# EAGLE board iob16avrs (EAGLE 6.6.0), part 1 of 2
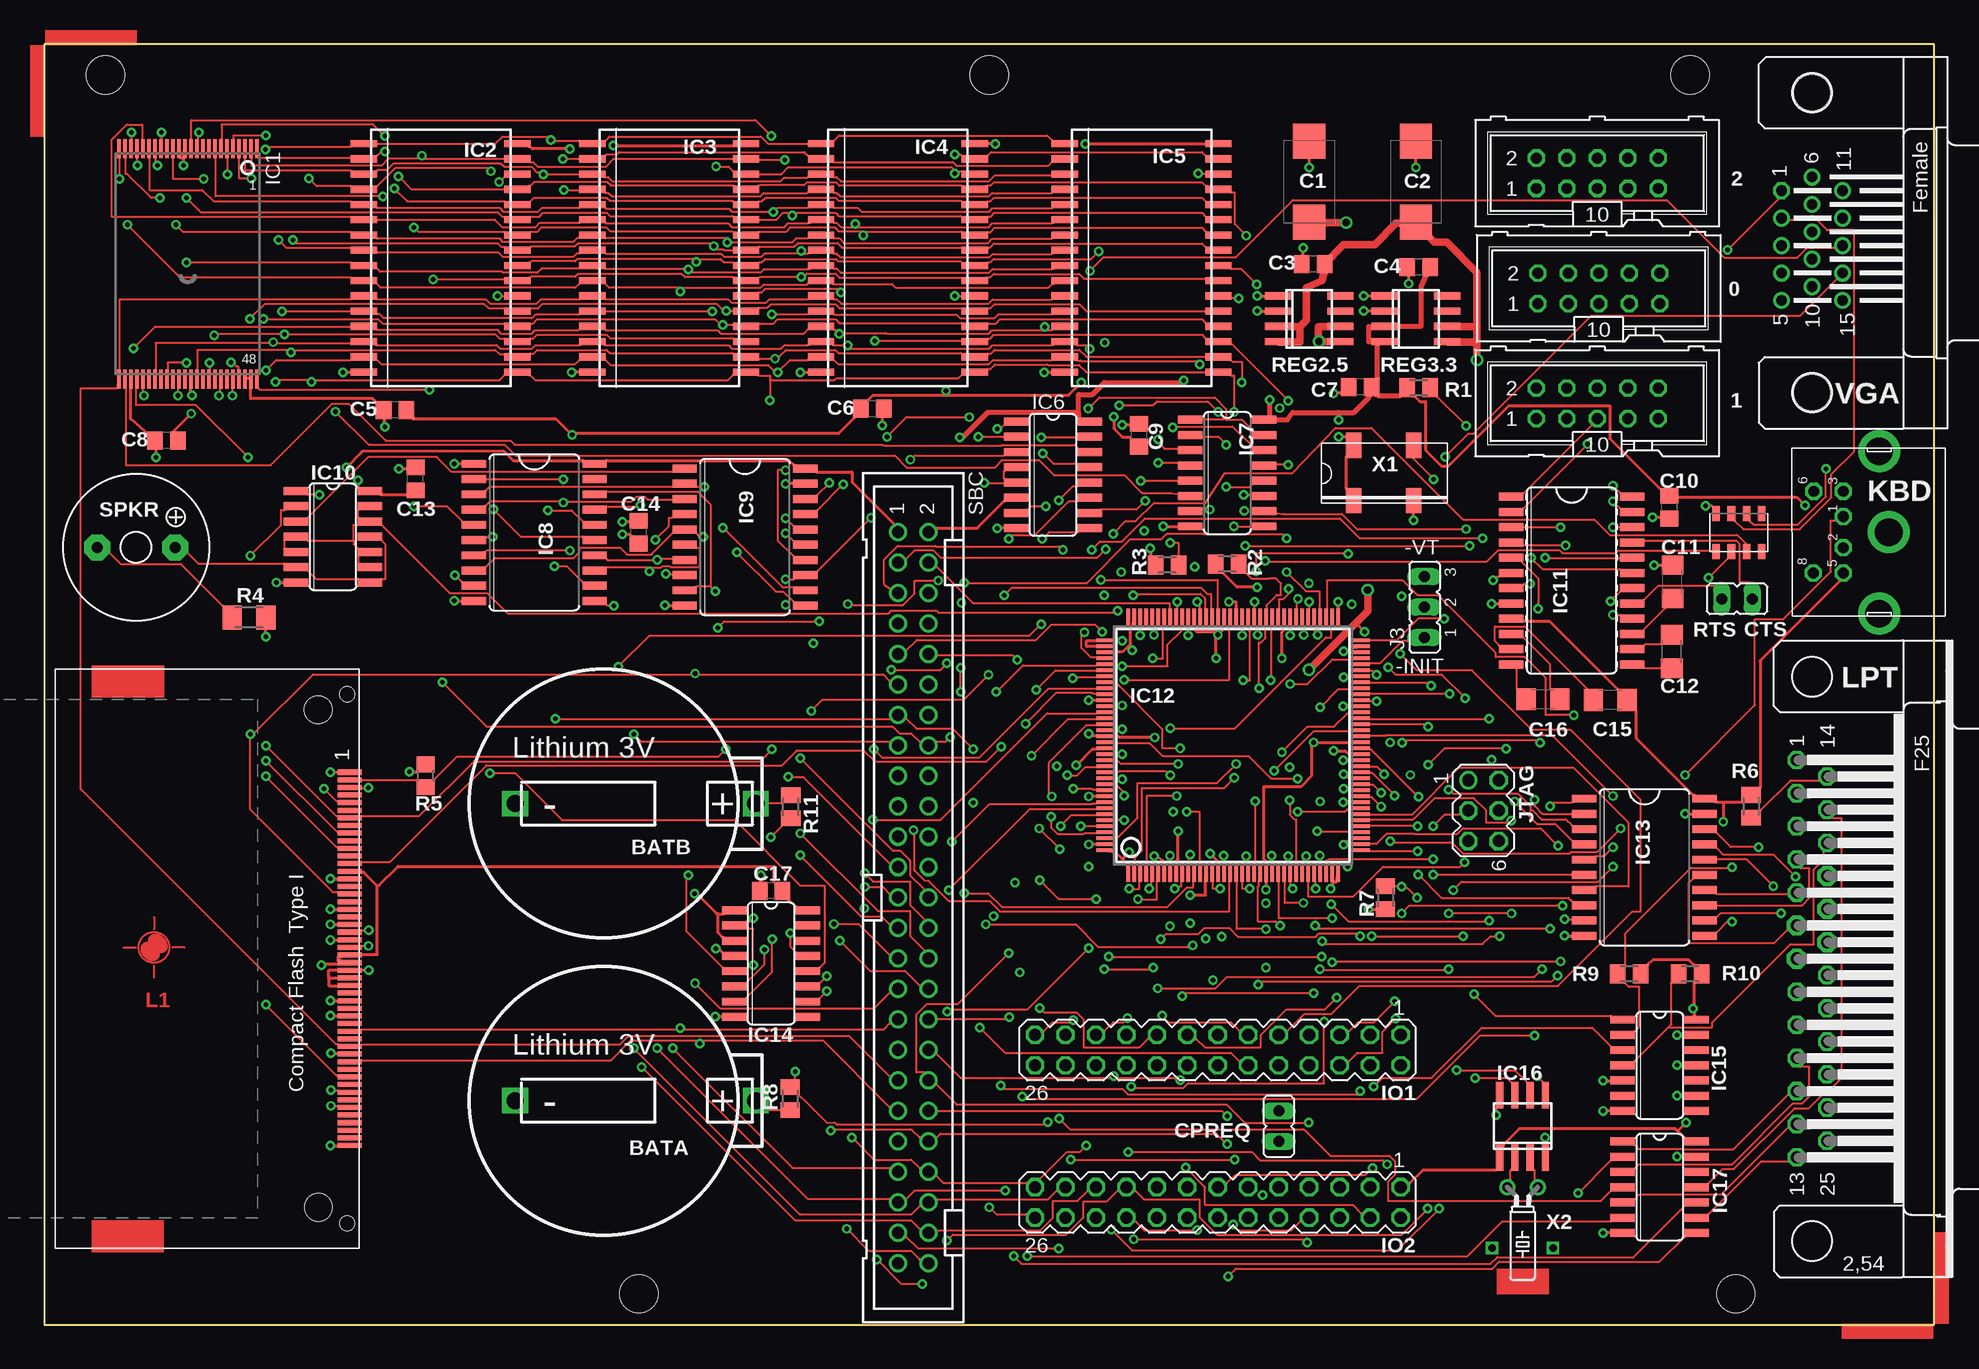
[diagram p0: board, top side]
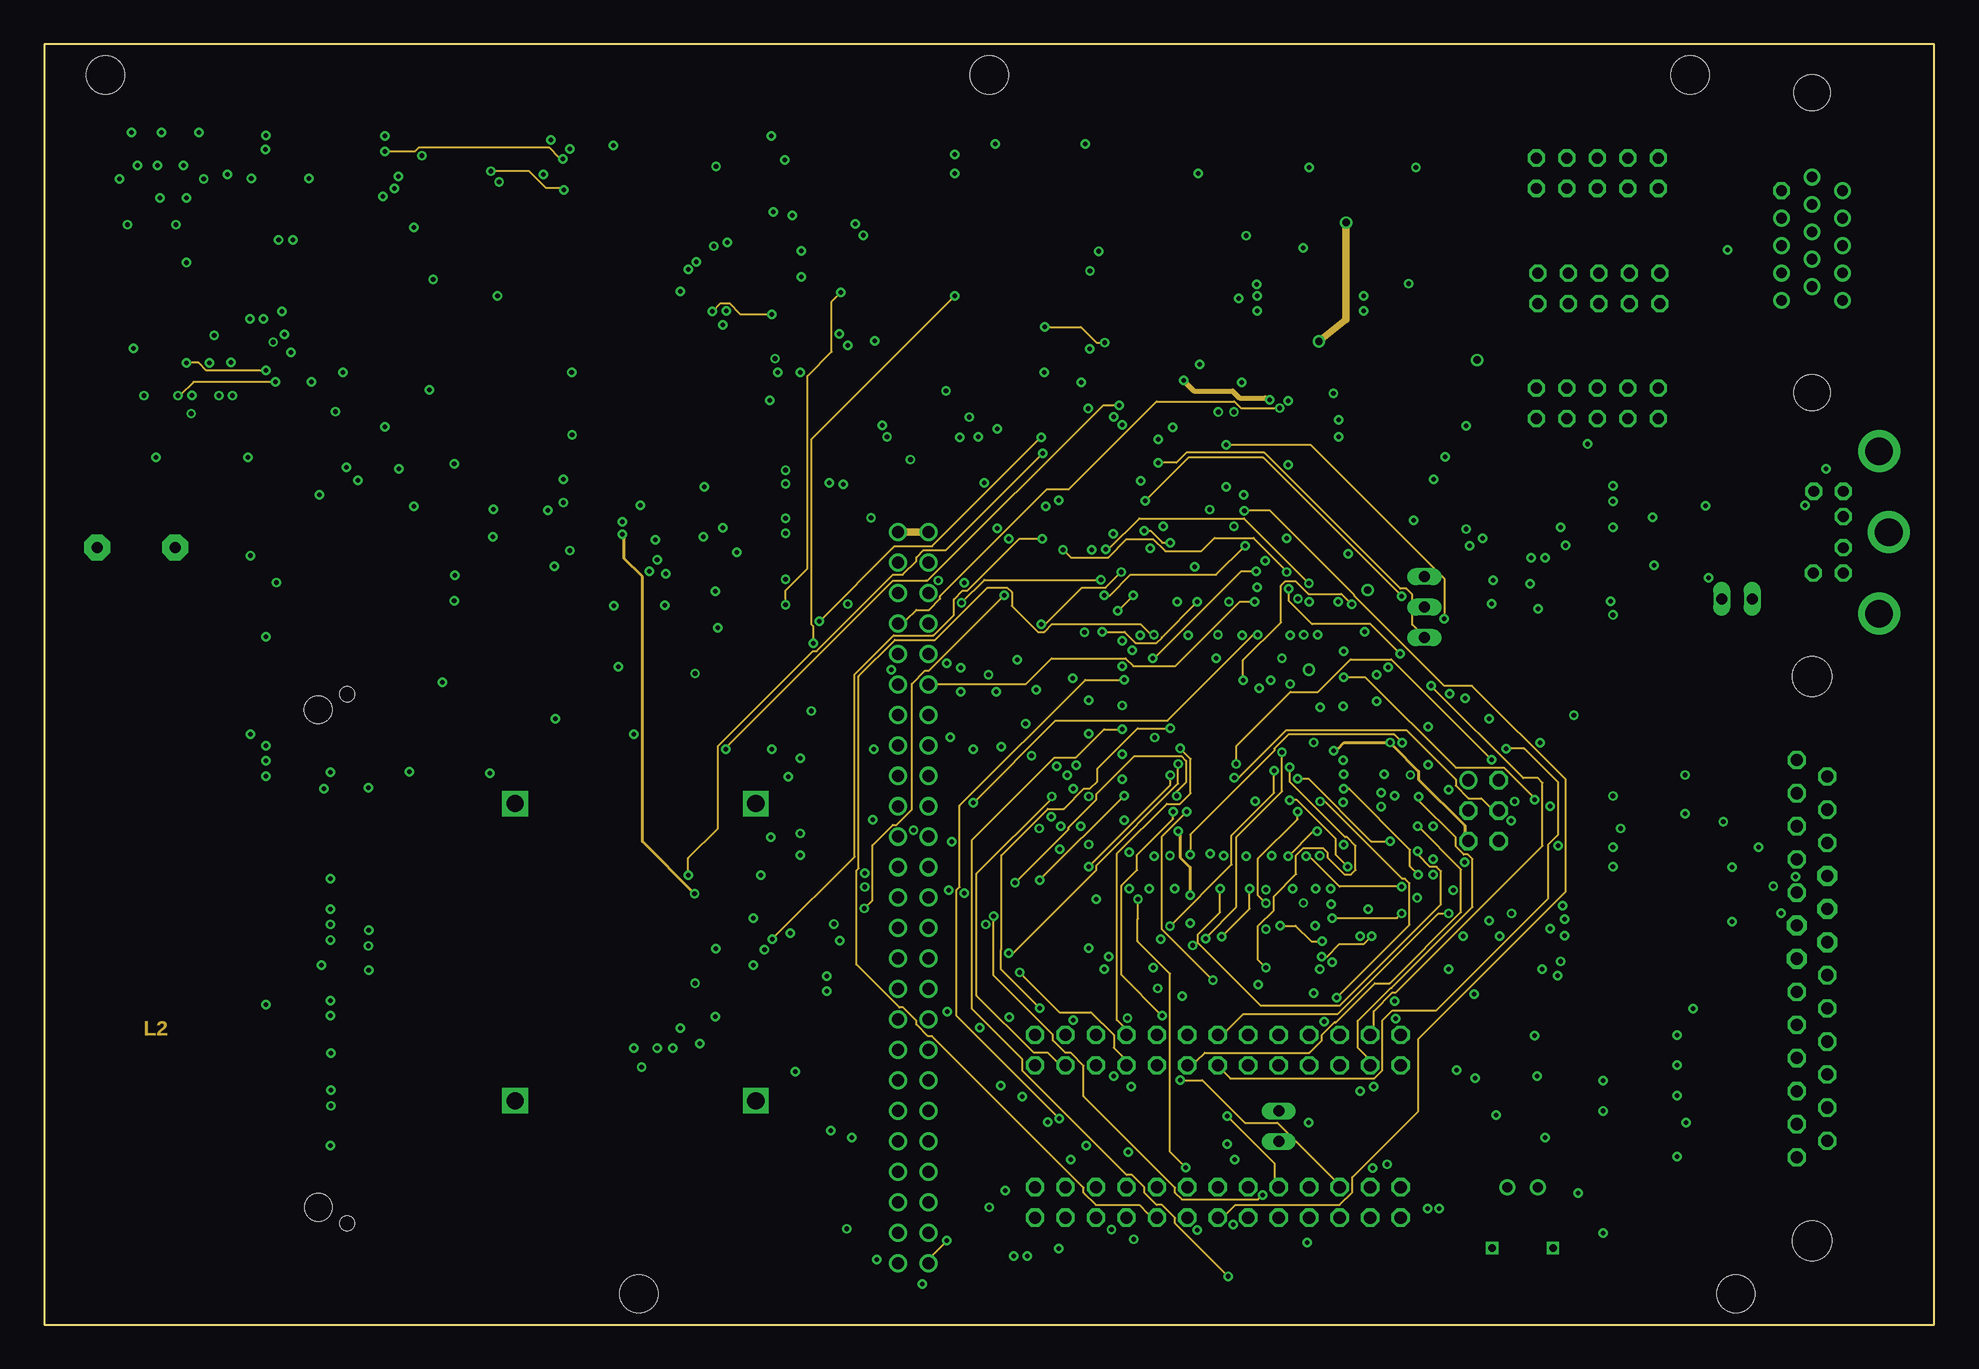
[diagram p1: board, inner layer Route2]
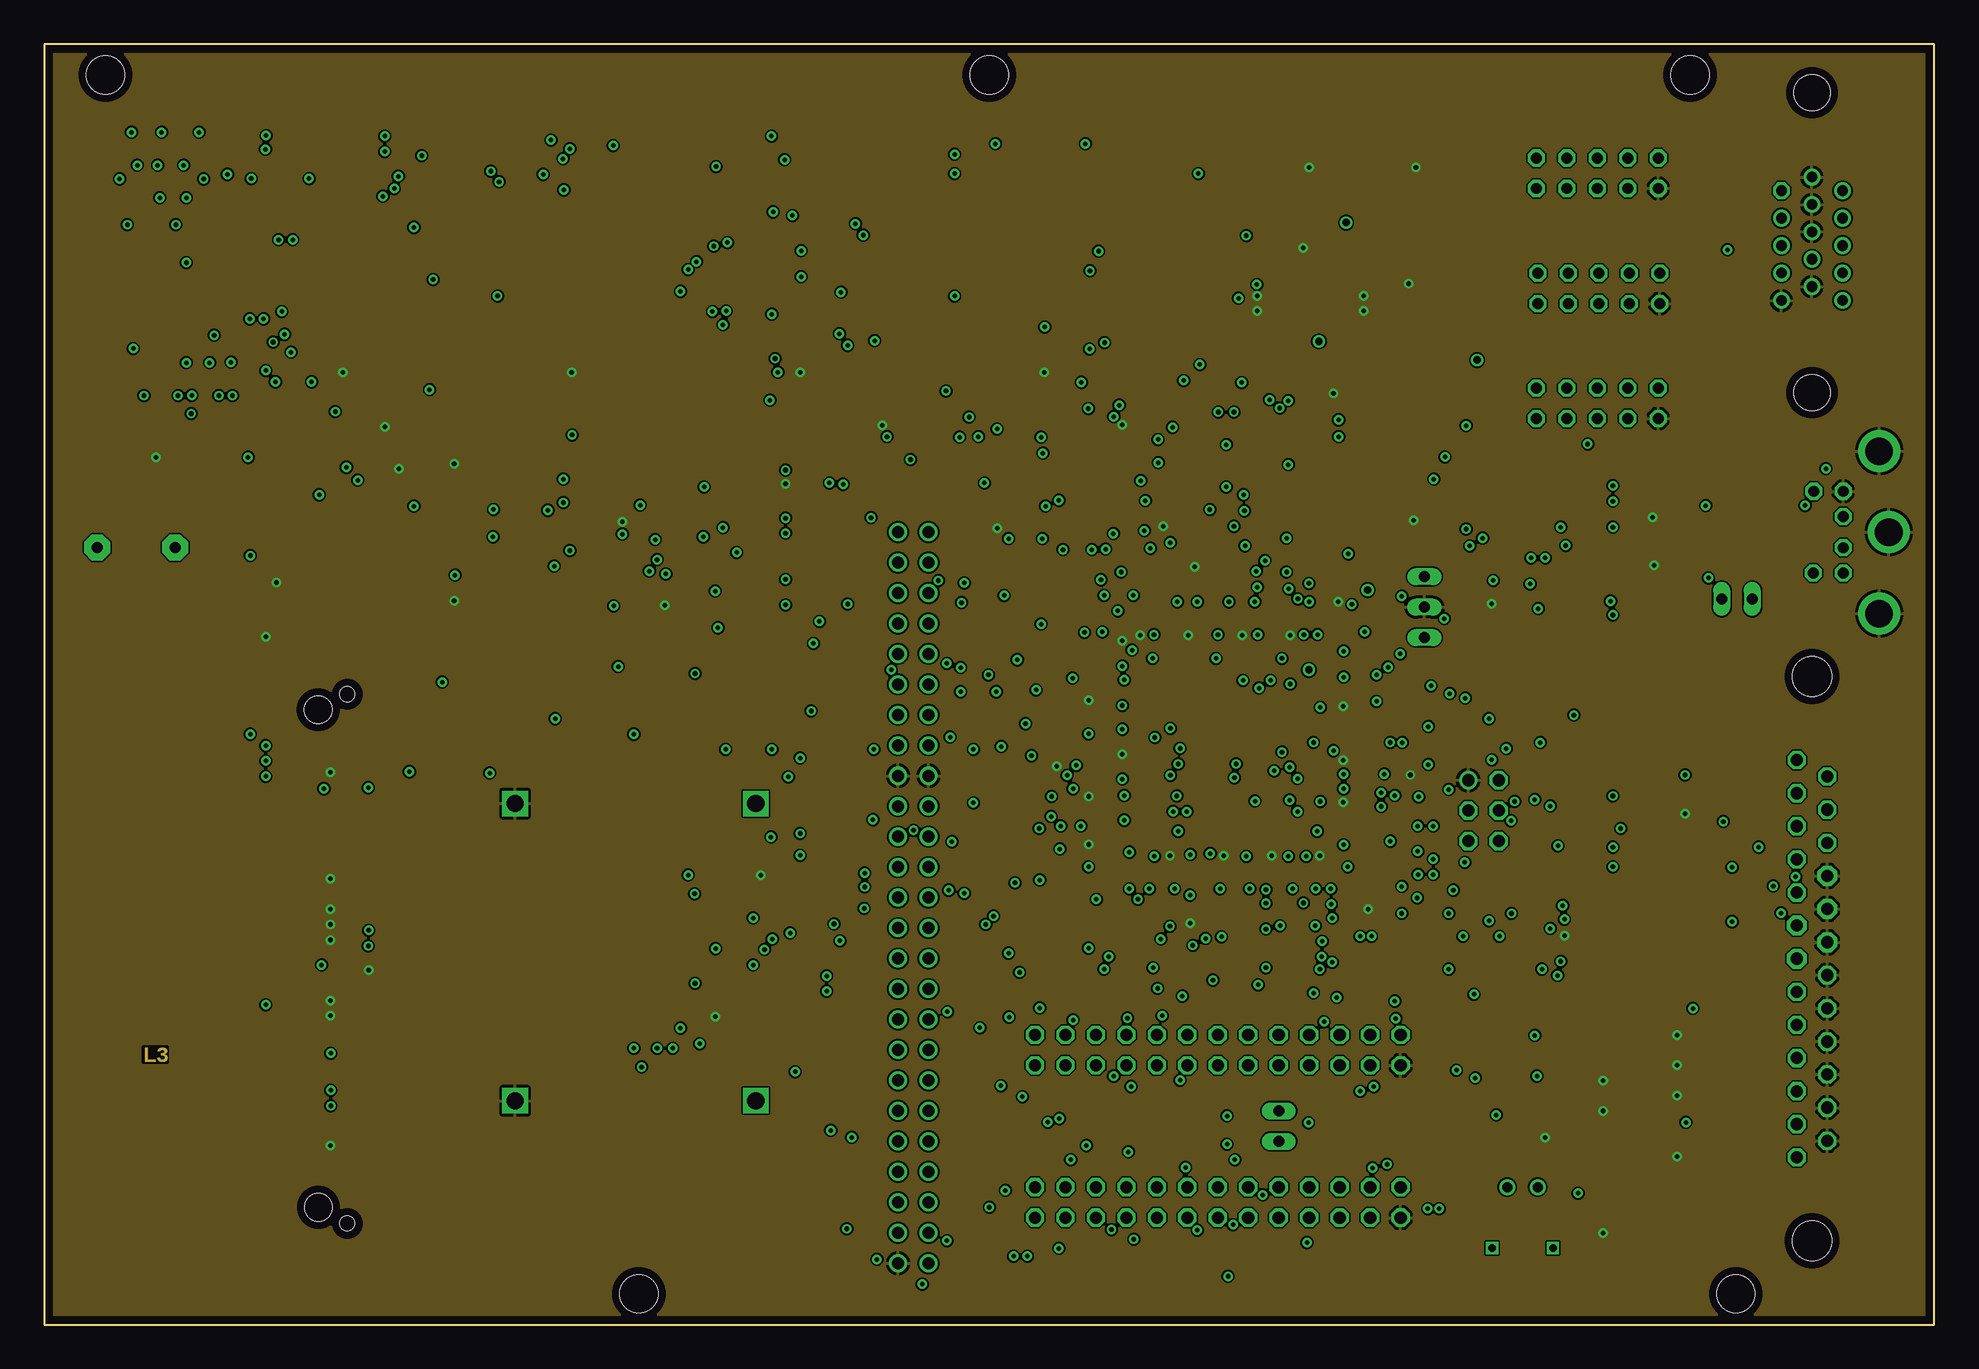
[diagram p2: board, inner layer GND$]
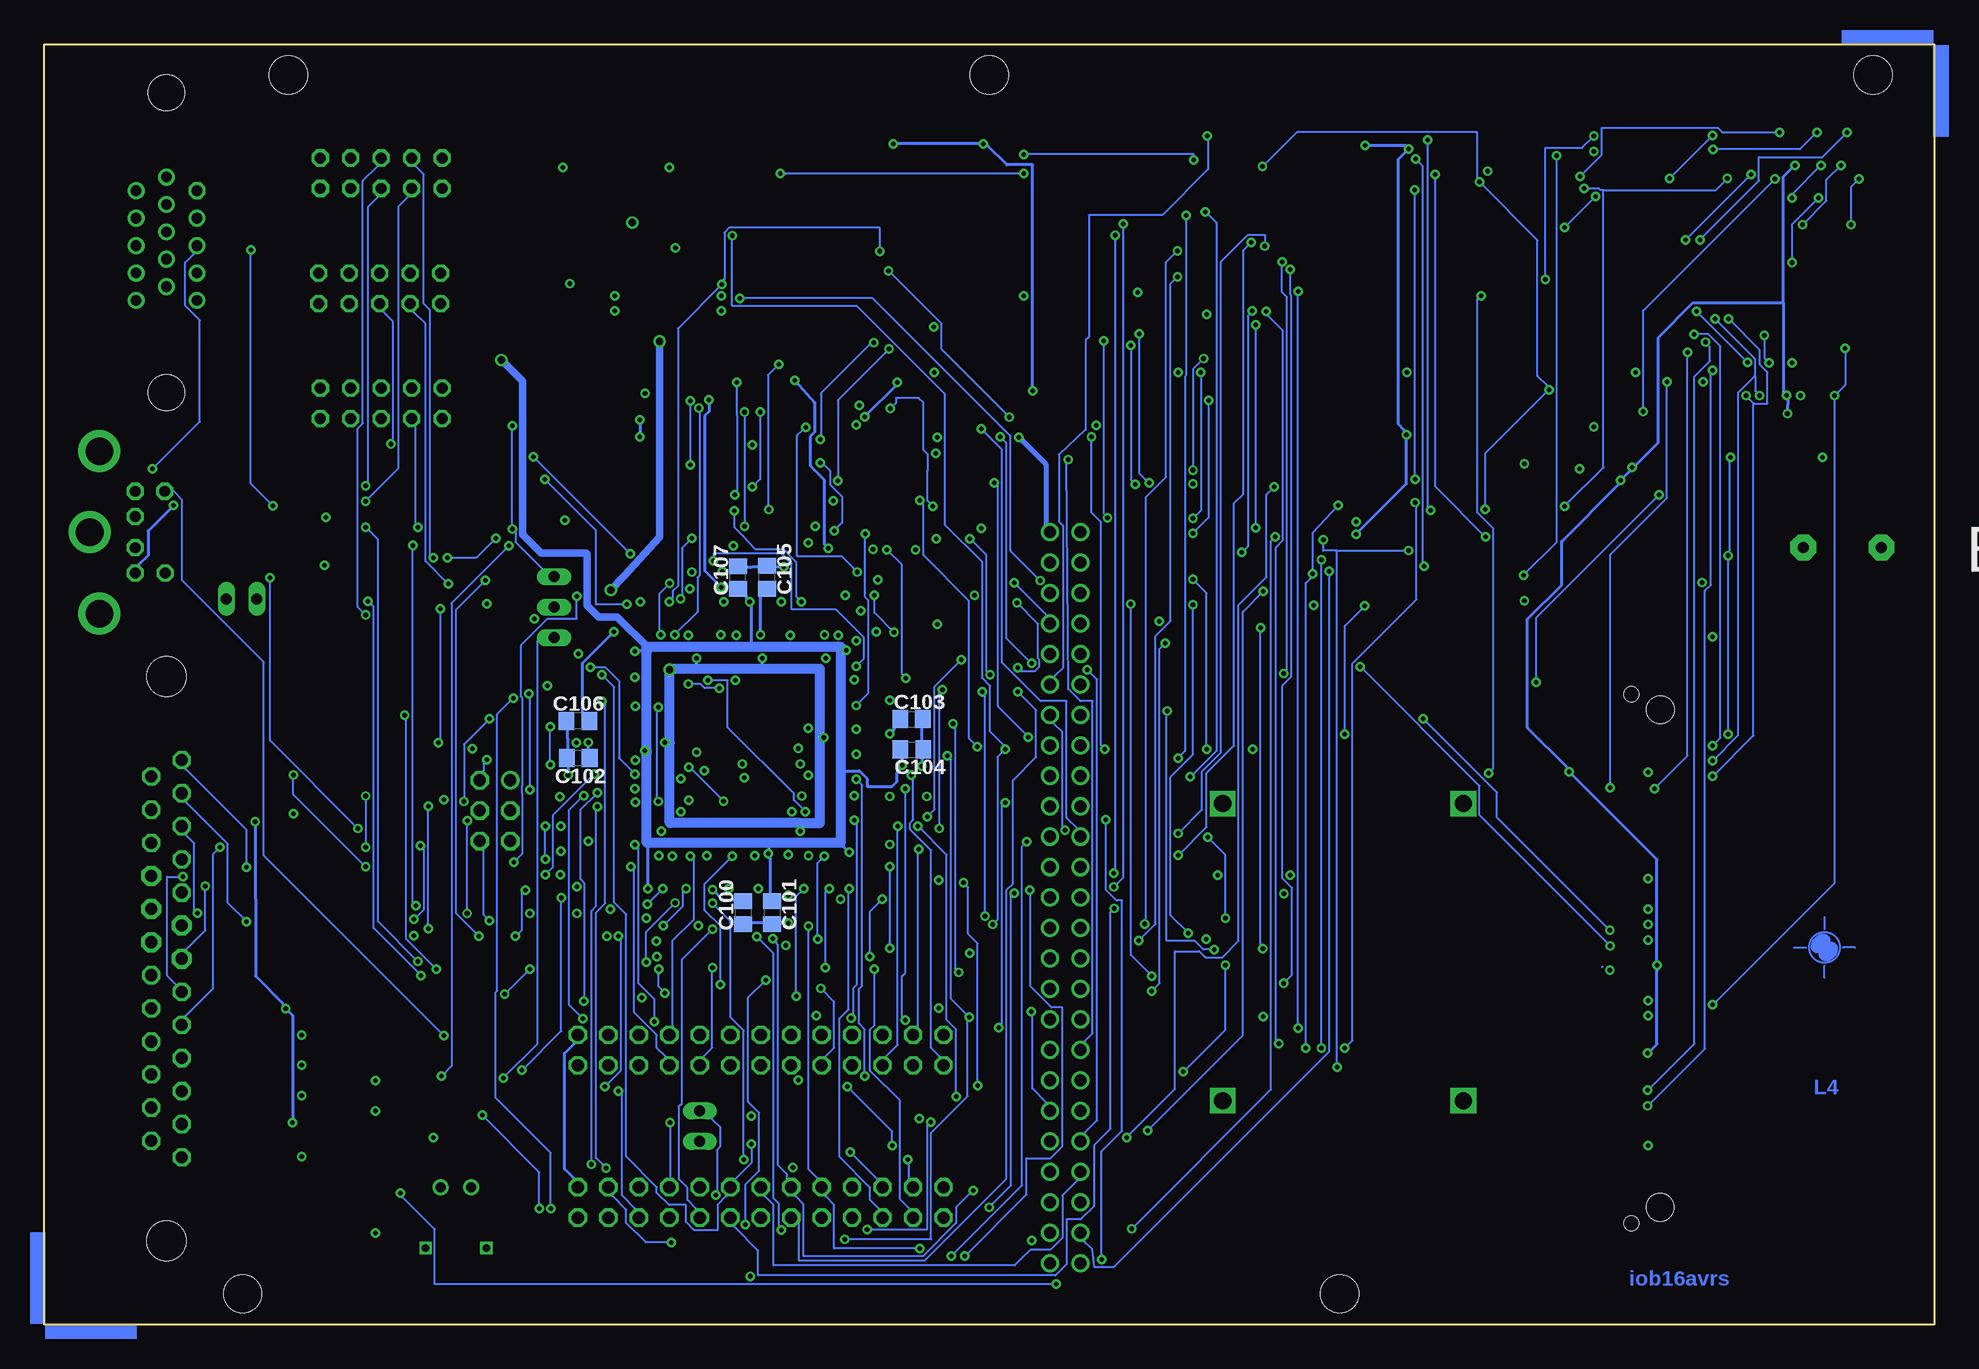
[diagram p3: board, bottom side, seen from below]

Size 157.53 x 106.73 mm. Coordinates in mm from the lower left corner, seen from the top.
Outline: 0,0 157.53,0 157.53,106.73 0,106.73 0,0
Copper layers (1*2*15*16): Top 0.035mm / dielectric 1.5mm / Route2 0.035mm / dielectric 0.15mm / GND$ 0.035mm / dielectric 0.2mm / Bottom 0.035mm
Design rules "iob *": minimum track width 7mil, minimum drill 15mil, track to track 6mil, track to pad 6mil, pad to pad 6mil, via to via 6mil, smd to smd 0mil, copper to edge 25mil, drill to drill 8mil, minimum pad ring 10mil, minimum via ring 8mil, stop-mask expansion 0mil, vias tented up to drill 20mil, thermal gap 10mil
Net classes: 1 power: width 0.254 mm, drill 0.381 mm, clearance 0.203 mm; 2 gnd: width 0.254 mm, drill 0.381 mm; 3 power2: width 0.254 mm, drill 0.381 mm
Holes 3.17 mm at 78.77,104.17 141,2.57 5.11,104.17 49.56,2.57 137.19,104.17

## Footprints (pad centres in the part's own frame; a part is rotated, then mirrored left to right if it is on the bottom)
CR2032HOLDER = drill 1.422 square: + 12.7,0; - -7.366,0
D/7343-31W = smd 2.95 x 2.7: + 3.375,0; - -3.375,0
C0805 = smd 1.3 x 1.5: 1 -0.95,0; 2 0.95,0
C1206 = smd 1.6 x 1.8: 1 -1.4,0; 2 1.4,0
CF_SOCKET2_SMT = smd 0.42 x 2: 1 15.545,-17.805; 2 14.275,-17.805; 3 13.005,-17.805; 4 11.735,-17.805; 5 10.465,-17.805; 6 9.195,-17.805; 7 7.925,-17.805; 8 6.655,-17.805; 9 5.385,-17.805; 10 4.115,-17.805; 11 2.845,-17.805; 12 1.575,-17.805; 13 0.305,-17.805; 14 -0.965,-17.805; 15 -2.235,-17.805; 16 -3.505,-17.805; 17 -4.775,-17.805; 18 -6.045,-17.805; 19 -7.315,-17.805; 20 -8.585,-17.805; 21 -9.855,-17.805; 22 -11.125,-17.805; 23 -12.395,-17.805; 24 -13.665,-17.805; 25 -14.935,-17.805; 26 14.91,-17.805; 27 13.64,-17.805; 28 12.37,-17.805; 29 11.1,-17.805; 30 9.83,-17.805; 31 8.56,-17.805; 32 7.29,-17.805; 33 6.02,-17.805; 34 4.75,-17.805; 35 3.48,-17.805; 36 2.21,-17.805; 37 0.94,-17.805; 38 -0.33,-17.805; 39 -1.6,-17.805; 40 -2.87,-17.805; 41 -4.14,-17.805; 42 -5.41,-17.805; 43 -6.68,-17.805; 44 -7.95,-17.805; 45 -9.22,-17.805; 46 -10.49,-17.805; 47 -11.76,-17.805; 48 -13.03,-17.805; 49 -14.3,-17.805; 50 -15.57,-17.805 | hole 2.3: 20.747,-15.177; -20.72,-15.208 | hole 1.27: -22.062,-17.6; 22.048,-17.6
JP1 = drill 0.914 long: 1 0,-1.27; 2 0,1.27
TSOP48 = smd 0.3 x 1.6: 1 -5.75,-9.6; 2 -5.25,-9.6; 3 -4.75,-9.6; 4 -4.25,-9.6; 5 -3.75,-9.6; 6 -3.25,-9.6; 7 -2.75,-9.6; 8 -2.25,-9.6; 9 -1.75,-9.6; 10 -1.25,-9.6; 11 -0.75,-9.6; 12 -0.25,-9.6; 13 0.25,-9.6; 14 0.75,-9.6; 15 1.25,-9.6; 16 1.75,-9.6; 17 2.25,-9.6; 18 2.75,-9.6; 19 3.25,-9.6; 20 3.75,-9.6; 21 4.25,-9.6; 22 4.75,-9.6; 23 5.25,-9.6; 24 5.75,-9.6; 25 5.75,9.6; 26 5.25,9.6; 27 4.75,9.6; 28 4.25,9.6; 29 3.75,9.6; 30 3.25,9.6; 31 2.75,9.6; 32 2.25,9.6; 33 1.75,9.6; 34 1.25,9.6; 35 0.75,9.6; 36 0.25,9.6; 37 -0.25,9.6; 38 -0.75,9.6; 39 -1.25,9.6; 40 -1.75,9.6; 41 -2.25,9.6; 42 -2.75,9.6; 43 -3.25,9.6; 44 -3.75,9.6; 45 -4.25,9.6; 46 -4.75,9.6; 47 -5.25,9.6; 48 -5.75,9.6
SOP32 = smd 0.6 x 2.2: 1 -9.525,-6.4; 2 -8.255,-6.4; 3 -6.985,-6.4; 4 -5.715,-6.4; 5 -4.445,-6.4; 6 -3.175,-6.4; 7 -1.905,-6.4; 8 -0.635,-6.4; 9 0.635,-6.4; 10 1.905,-6.4; 11 3.175,-6.4; 12 4.445,-6.4; 13 5.715,-6.4; 14 6.985,-6.4; 15 8.255,-6.4; 16 9.525,-6.4; 17 9.525,6.4; 18 8.255,6.4; 19 6.985,6.4; 20 5.715,6.4; 21 4.445,6.4; 22 3.175,6.4; 23 1.905,6.4; 24 0.635,6.4; 25 -0.635,6.4; 26 -1.905,6.4; 27 -3.175,6.4; 28 -4.445,6.4; 29 -5.715,6.4; 30 -6.985,6.4; 31 -8.255,6.4; 32 -9.525,6.4
SO16 = smd 0.66 x 2.032: 1 -4.445,-3.073; 2 -3.175,-3.073; 3 -1.905,-3.073; 4 -0.635,-3.073; 5 0.635,-3.073; 6 1.905,-3.073; 7 3.175,-3.073; 8 4.445,-3.073; 9 4.445,3.073; 10 3.175,3.073; 11 1.905,3.073; 12 0.635,3.073; 13 -0.635,3.073; 14 -1.905,3.073; 15 -3.175,3.073; 16 -4.445,3.073
SO20W = smd 0.66 x 2.032: 1 -5.715,-5.029; 2 -4.445,-5.029; 3 -3.175,-5.029; 4 -1.905,-5.029; 5 -0.635,-5.029; 6 0.635,-5.029; 7 1.905,-5.029; 8 3.175,-5.029; 9 4.445,-5.029; 10 5.715,-5.029; 11 5.715,5.029; 12 4.445,5.029; 13 3.175,5.029; 14 1.905,5.029; 15 0.635,5.029; 16 -0.635,5.029; 17 -1.905,5.029; 18 -3.175,5.029; 19 -4.445,5.029; 20 -5.715,5.029
SO14 = smd 0.66 x 2.032: 1 -3.81,-3.073; 2 -2.54,-3.073; 3 -1.27,-3.073; 4 0,-3.073; 5 1.27,-3.073; 6 2.54,-3.073; 7 3.81,-3.073; 8 3.81,3.073; 9 2.54,3.073; 10 1.27,3.073; 11 0,3.073; 12 -1.27,3.073; 13 -2.54,3.073; 14 -3.81,3.073
SO24L = smd 0.66 x 2.032: 1 -6.985,-5.029; 2 -5.715,-5.029; 3 -4.445,-5.029; 4 -3.175,-5.029; 5 -1.905,-5.029; 6 -0.635,-5.029; 7 0.635,-5.029; 8 1.905,-5.029; 9 3.175,-5.029; 10 4.445,-5.029; 11 5.715,-5.029; 12 6.985,-5.029; 13 6.985,5.029; 14 5.715,5.029; 15 4.445,5.029; 16 3.175,5.029; 17 1.905,5.029; 18 0.635,5.029; 19 -0.635,5.029; 20 -1.905,5.029; 21 -3.175,5.029; 22 -4.445,5.029; 23 -5.715,5.029; 24 -6.985,5.029
TQFP144 = smd 0.3 x 1.6: 1 -8.75,-10.6; 2 -8.25,-10.6; 3 -7.75,-10.6; 4 -7.25,-10.6; 5 -6.75,-10.6; 6 -6.25,-10.6; 7 -5.75,-10.6; 8 -5.25,-10.6; 9 -4.75,-10.6; 10 -4.25,-10.6; 11 -3.75,-10.6; 12 -3.25,-10.6; 13 -2.75,-10.6; 14 -2.25,-10.6; 15 -1.75,-10.6; 16 -1.25,-10.6; 17 -0.75,-10.6; 18 -0.25,-10.6; 19 0.25,-10.6; 20 0.75,-10.6; 21 1.25,-10.6; 22 1.75,-10.6; 23 2.25,-10.6; 24 2.75,-10.6; 25 3.25,-10.6; 26 3.75,-10.6; 27 4.25,-10.6; 28 4.75,-10.6; 29 5.25,-10.6; 30 5.75,-10.6; 31 6.25,-10.6; 32 6.75,-10.6; 33 7.25,-10.6; 34 7.75,-10.6; 35 8.25,-10.6; 36 8.75,-10.6; 73 8.75,10.6; 74 8.25,10.6; 75 7.75,10.6; 76 7.25,10.6; 77 6.75,10.6; 78 6.25,10.6; 79 5.75,10.6; 80 5.25,10.6; 81 4.75,10.6; 82 4.25,10.6; 83 3.75,10.6; 84 3.25,10.6; 85 2.75,10.6; 86 2.25,10.6; 87 1.75,10.6; 88 1.25,10.6; 89 0.75,10.6; 90 0.25,10.6; 91 -0.25,10.6; 92 -0.75,10.6; 93 -1.25,10.6; 94 -1.75,10.6; 95 -2.25,10.6; 96 -2.75,10.6; 97 -3.25,10.6; 98 -3.75,10.6; 99 -4.25,10.6; 100 -4.75,10.6; 101 -5.25,10.6; 102 -5.75,10.6; 103 -6.25,10.6; 104 -6.75,10.6; 105 -7.25,10.6; 106 -7.75,10.6; 107 -8.25,10.6; 108 -8.75,10.6 | smd 1.6 x 0.3: 37 10.6,-8.75; 38 10.6,-8.25; 39 10.6,-7.75; 40 10.6,-7.25; 41 10.6,-6.75; 42 10.6,-6.25; 43 10.6,-5.75; 44 10.6,-5.25; 45 10.6,-4.75; 46 10.6,-4.25; 47 10.6,-3.75; 48 10.6,-3.25; 49 10.6,-2.75; 50 10.6,-2.25; 51 10.6,-1.75; 52 10.6,-1.25; 53 10.6,-0.75; 54 10.6,-0.25; 55 10.6,0.25; 56 10.6,0.75; 57 10.6,1.25; 58 10.6,1.75; 59 10.6,2.25; 60 10.6,2.75; 61 10.6,3.25; 62 10.6,3.75; 63 10.6,4.25; 64 10.6,4.75; 65 10.6,5.25; 66 10.6,5.75; 67 10.6,6.25; 68 10.6,6.75; 69 10.6,7.25; 70 10.6,7.75; 71 10.6,8.25; 72 10.6,8.75; 109 -10.6,8.75; 110 -10.6,8.25; 111 -10.6,7.75; 112 -10.6,7.25; 113 -10.6,6.75; 114 -10.6,6.25; 115 -10.6,5.75; 116 -10.6,5.25; 117 -10.6,4.75; 118 -10.6,4.25; 119 -10.6,3.75; 120 -10.6,3.25; 121 -10.6,2.75; 122 -10.6,2.25; 123 -10.6,1.75; 124 -10.6,1.25; 125 -10.6,0.75; 126 -10.6,0.25; 127 -10.6,-0.25; 128 -10.6,-0.75; 129 -10.6,-1.25; 130 -10.6,-1.75; 131 -10.6,-2.25; 132 -10.6,-2.75; 133 -10.6,-3.25; 134 -10.6,-3.75; 135 -10.6,-4.25; 136 -10.6,-4.75; 137 -10.6,-5.25; 138 -10.6,-5.75; 139 -10.6,-6.25; 140 -10.6,-6.75; 141 -10.6,-7.25; 142 -10.6,-7.75; 143 -10.6,-8.25; 144 -10.6,-8.75
SO08 = smd 0.6 x 2.2: 1 -1.905,-2.6; 2 -0.635,-2.6; 3 0.635,-2.6; 4 1.905,-2.6; 5 1.905,2.6; 6 0.635,2.6; 7 -0.635,2.6; 8 -1.905,2.6
MA13-2 = drill 1.016 octagon: 1 -15.24,-1.27; 2 -15.24,1.27; 3 -12.7,-1.27; 4 -12.7,1.27; 5 -10.16,-1.27; 6 -10.16,1.27; 7 -7.62,-1.27; 8 -7.62,1.27; 9 -5.08,-1.27; 10 -5.08,1.27; 11 -2.54,-1.27; 12 -2.54,1.27; 13 0,-1.27; 14 0,1.27; 15 2.54,-1.27; 16 2.54,1.27; 17 5.08,-1.27; 18 5.08,1.27; 19 7.62,-1.27; 20 7.62,1.27; 21 10.16,-1.27; 22 10.16,1.27; 23 12.7,-1.27; 24 12.7,1.27; 25 15.24,-1.27; 26 15.24,1.27
JP2 = drill 0.914 long: 1 -2.54,0; 2 0,0; 3 2.54,0
MA03-2 = drill 1.016: 1 -2.54,-1.27 | drill 1.016 octagon: 2 -2.54,1.27; 3 0,-1.27; 4 0,1.27; 5 2.54,-1.27; 6 2.54,1.27
M_DIN6 = drill 0.9 pad 1.422 octagon: 1 -1.3,-3.75; 2 1.3,-3.75; 3 -3.4,-3.75; 5 3.4,-3.75; 6 -3.4,-6.2; 8 3.4,-6.25 | drill 2.3 pad 3.5: SH1 6.8,-0.75; SH2 0,0.05; SH3 -6.75,-0.75
F25H = drill 1.016 octagon: 1 -16.561,-1.27; 2 -13.792,-1.27; 3 -11.049,-1.27; 4 -8.28,-1.27; 5 -5.512,-1.27; 8 2.769,-1.27; 9 5.512,-1.27; 10 8.28,-1.27; 11 11.049,-1.27; 12 13.792,-1.27; 13 16.561,-1.27; 14 -15.189,1.27; 15 -12.421,1.27; 16 -9.652,1.27; 20 1.372,1.27; 21 4.14,1.27; 22 6.909,1.27; 23 9.652,1.27; 24 12.421,1.27; 25 15.189,1.27 | drill 1.016 pad 1.67 octagon: 6 -2.769,-1.27; 7 0,-1.27; 17 -6.909,1.27; 18 -4.14,1.27; 19 -1.372,1.27 | hole 3.302: -23.52,0; 23.52,0
M0805 = smd 1.3 x 1.6: 1 -0.95,0; 2 0.95,0
M1206 = smd 1.6 x 2: 1 -1.4,0; 2 1.4,0
R0805 = smd 1.3 x 1.5: 1 -0.95,0; 2 0.95,0
RN-CTS-744C043 = smd 0.635 x 1.27: 1 -1.905,-1.905; 2 -0.635,-1.905; 3 0.635,-1.905; 4 1.905,-1.905; 5 1.905,1.27; 6 0.635,1.27; 7 -0.635,1.27; 8 -1.905,1.27
PAK100/2500-50 = drill 1 pad 1.422: 1 -30.48,-1.27; 2 -30.48,1.27; 3 -27.94,-1.27; 4 -27.94,1.27; 5 -25.4,-1.27; 6 -25.4,1.27; 7 -22.86,-1.27; 8 -22.86,1.27; 9 -20.32,-1.27; 10 -20.32,1.27; 11 -17.78,-1.27; 12 -17.78,1.27; 13 -15.24,-1.27; 14 -15.24,1.27; 15 -12.7,-1.27; 16 -12.7,1.27; 17 -10.16,-1.27; 18 -10.16,1.27; 19 -7.62,-1.27; 20 -7.62,1.27; 21 -5.08,-1.27; 22 -5.08,1.27; 23 -2.54,-1.27; 24 -2.54,1.27; 25 0,-1.27; 26 0,1.27; 27 2.54,-1.27; 28 2.54,1.27; 29 5.08,-1.27; 30 5.08,1.27; 31 7.62,-1.27; 32 7.62,1.27; 33 10.16,-1.27; 34 10.16,1.27; 35 12.7,-1.27; 36 12.7,1.27; 37 15.24,-1.27; 38 15.24,1.27; 39 17.78,-1.27; 40 17.78,1.27; 41 20.32,-1.27; 42 20.32,1.27; 43 22.86,-1.27; 44 22.86,1.27; 45 25.4,-1.27; 46 25.4,1.27; 47 27.94,-1.27; 48 27.94,1.27; 49 30.48,-1.27; 50 30.48,1.27
ML10 = drill 0.914 octagon: 1 -5.08,-1.27; 2 -5.08,1.27; 3 -2.54,-1.27; 4 -2.54,1.27; 5 0,-1.27; 6 0,1.27; 7 2.54,-1.27; 8 2.54,1.27; 9 5.08,-1.27; 10 5.08,1.27
KSS1201 = drill 0.914 pad 2.159 octagon: + 3.251,0; - -3.251,0
HDF15H = drill 0.9 octagon: 1 4.329,2.54 | drill 0.9: 2 2.043,2.54; 3 -0.243,2.54; 4 -2.529,2.54; 5 -4.815,2.54; 6 5.472,0; 7 3.186,0; 8 0.9,0; 9 -1.386,0; 10 -3.672,0; 11 4.329,-2.54; 12 2.043,-2.54; 13 -0.243,-2.54; 14 -2.529,-2.54; 15 -4.815,-2.54 | hole 3: -12.5,0; 12.5,0
SG636 = smd 1.3 x 2.1: P$1 0,0; P$2 5,0; P$3 5,4.6; P$4 0,4.6
TC26H = drill 0.813: 1 -1.27,0; 2 1.27,0

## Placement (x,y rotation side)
BATA  CR2032  [CR2032HOLDER]  46.61,18.67 0 top
BATB  CR2032  [CR2032HOLDER]  46.61,43.43 0 top
C1  10u  [D/7343-31W]  105.44,95.28 270 top
C2  10u  [D/7343-31W]  114.33,95.28 270 top
C3  0u1  [C0805]  105.77,88.39 180 top
C4  0u1  [C0805]  114.55,88.16 180 top
C5  0u1  [C0805]  29.24,76.23 180 top
C6  0u1  [C0805]  69.01,76.35 0 top
C7  0u1  [C0805]  109.68,78.16 180 top
C8  0u1  [C0805]  10.19,73.69 180 top
C9  0u1  [C0805]  91.26,74.14 90 top
C10  0u1  [C0805]  135.43,68.15 270 top
C11  0.1uF  [C1206]  135.71,61.93 90 top
C12  0.1uF  [C1206]  135.66,56.11 90 top
C13  0u1  [C0805]  30.94,70.51 90 top
C14  0u1  [C0805]  49.56,66.07 90 top
C15  0.1uF  [C1206]  130.53,52.07 180 top
C16  0.1uF  [C1206]  124.92,52.12 180 top
C17  0u1  [C0805]  60.58,36.17 180 top
C100  0u1  [C0805]  99.29,34.34 270 bottom
C101  0u1  [C0805]  96.88,34.34 270 bottom
C102  0u1  [C0805]  113.03,47.22 180 bottom
C103  0u1  [C0805]  85.24,50.47 0 bottom
C104  0u1  [C0805]  85.22,47.93 0 bottom
C105  0u1  [C0805]  97.28,62.31 90 bottom
C106  0u1  [C0805]  113.06,50.32 180 bottom
C107  0u1  [C0805]  99.72,62.28 90 bottom
CF1  CF_CMM_SOCKET2  [CF_SOCKET2_SMT]  7.65,30.51 90 top
CPREQ  [JP1]  102.9,16.54 0 top
HS2  [JP1]  141.1,60.5 270 top
IC1  28F400E  [TSOP48]  11.96,88.43 180 top
IC2  628512  [SOP32]  33.05,88.93 270 top
IC3  628512  [SOP32]  52.1,88.93 270 top
IC4  628512  [SOP32]  71.15,88.93 270 top
IC5  628512  [SOP32]  91.47,88.93 270 top
IC6  74AHC138D  [SO16]  84.07,70.84 270 top
IC7  74HC367D  [SO16]  98.6,70.99 270 top
IC8  74ACT373DW  [SO20W]  40.84,66.04 270 top
IC9  74ACT245DW  [SO20W]  58.39,65.66 270 top
IC10  74ACT32D  [SO14]  24.05,65.68 270 top
IC11  MAX208ECWG  [SO24L]  127.3,62.03 270 top
IC12  XC2S100-5TQ144C  [TQFP144]  99.09,48.29 0 top
IC13  74ACT245DW  [SO20W]  133.38,38.13 270 top
IC14  DS1321D  [SO16]  60.58,30.1 270 top
IC15  74ACT05D  [SO14]  134.65,21.62 270 top
IC16  DS1302  [SO08]  123.22,16.54 0 top
IC17  74ACT04D  [SO14]  134.65,11.46 270 top
IO1  [MA13-2]  97.82,22.89 180 top
IO2  [MA13-2]  97.82,10.19 180 top
J3  [JP2]  115.04,59.82 90 top
JTAG  [MA03-2]  119.96,42.85 270 top
KBD  [M_DIN6]  153.7,66.07 270 top
LPT  [F25H]  147.35,30.51 270 top
R1  10K  [M0805]  114.55,78.11 180 top
R2  10K  [M0805]  98.6,63.4 0 top
R3  10K  [M0805]  93.6,63.32 0 top
R4  100ohm  [M1206]  17.07,58.95 0 top
R5  10K  [R0805]  31.78,45.75 90 top
R6  4K7  [M0805]  142.27,43.21 90 top
R7  10K  [M0805]  111.79,35.59 90 top
R8  470ohm  [M0805]  62.15,18.85 90 top
R9  4K7  [M0805]  132.11,29.24 0 top
R10  4K7  [M0805]  137.19,29.24 0 top
R11  470ohm  [M0805]  62.23,43.18 270 top
REG2.5  TPS77725D  [SO08]  105.44,83.85 270 top
REG3.3  TPS77733D  [SO08]  114.33,83.85 270 top
RN2  RN2  [RN-CTS-744C043]  141.25,66.34 0 top
SBC  2550-  [PAK100/2500-50]  72.42,35.6 270 top
SER1  [ML10]  129.44,95.99 0 top
SER2  [ML10]  129.57,86.39 0 top
SER3  [ML10]  129.44,76.81 0 top
SPKR  KSS1201  [KSS1201]  7.65,64.8 0 top
U$34  [PASS-ROUND]  9.14,31.45 0 top
U$42  [ANGLE-ARROW-NW1-16]  0.08,106.65 0 top
U$43  [ANGLE-ARROW-SE1-16]  157.45,0.08 0 top
VGA  [HDF15H]  147.35,90.2 90 top
X1  29.4912MHz  [SG636]  109.14,68.71 0 top
X2  32768  [TC26H]  123.22,11.46 180 top

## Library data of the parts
BATA BATB CF1 IC2-IC5 IC12 IC16 REG2.5 REG3.3 RN2 X1 = parts
C1-C17 C100-C107 R1-R11 = rcl
CPREQ HS2 J3 = jumper
IC1 = am29-memory
IC6 IC8-IC10 IC13 IC15 IC17 = 74xx-us
IC7 = 74xx-eu
IC11 = maxim; MPN: MAX208ECWG+; OC_FARNELL: unknown; OC_NEWARK: 67K4386
IC14 = ds1321
IO1 IO2 JTAG = con-lstb; OC_FARNELL: unknown; OC_NEWARK: unknown
KBD = mini_din
LPT VGA = con-subd; OC_FARNELL: unknown; OC_NEWARK: unknown
SBC = con-3m; OC_FARNELL: unknown; OC_NEWARK: unknown
SER1-SER3 = con-harting-ml; OC_FARNELL: unknown; OC_NEWARK: unknown
SPKR = buzzer; OC_FARNELL: unknown; OC_NEWARK: unknown
U$34 U$42 U$43 = marks
X2 = crystal; OC_FARNELL: unknown; OC_NEWARK: unknown

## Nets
2V5 [power2]: C1.+ C100.1 C103.1 C105.1 C106.1 IC12.9 IC12.14 IC12.24 IC12.55 IC12.82 IC12.92 IC12.97 IC12.125 REG2.5.5 REG2.5.6
5V [power]: C4.1 C7.1 C8.1 C10.1 C13.1 C15.1 C17.1 CF1.13 CF1.32 CF1.38 CF1.44 IC1.13 IC1.14 IC1.37 IC6.6 IC6.16 IC7.16 IC8.20 IC9.20 IC10.14 IC11.9 IC13.20 IC14.16 IC15.14 IC16.1 IC17.14 IO1.1 IO2.1 KBD.5 R1.2 R2.1 R3.1 R5.2 R6.2 R9.2 R10.2 REG3.3.3 REG3.3.4 SBC.1 SBC.2 X1.P$1 X1.P$4
B0: IC12.120 RN2.3
C0_L: IC12.79 SBC.7
C1_L: IC12.80 SBC.8
CF_DETECT_L: CF1.26 IC7.12 R5.1
CF_L: CF1.7 IC6.12
CF_READY: CF1.37 IC7.14
CPUDX0: IC12.122 IO2.3 SBC.34
CPUDX1: IC12.132 IO2.5 SBC.36
CPUDX2: IC12.129 IO2.7 SBC.38
CPUDX3: IC12.131 IO2.9 SBC.40
CPUDX4: IC8.18 IC9.9 IC12.67 IO2.11 SBC.42
CPUDX5: IC8.17 IC9.8 IC12.62 IO2.13 SBC.43
CPUDX6: IC8.14 IC9.7 IC12.60 IO2.15 SBC.45
CPUDX7: IC8.13 IC9.6 IC12.57 IO2.17 SBC.47
CPUDX8: IC8.8 IC9.5 IC12.49 IO2.19 SBC.50
CPUDX9: IC8.7 IC9.4 IC12.46 IO2.21 SBC.48
CPUDX10: IC8.4 IC9.3 IC12.44 IO2.23 SBC.46
CPUDX11: IC8.3 IC9.2 IC12.39 IO2.25 SBC.44
CTS2: HS2.1 IC11.17
DA0: IC1.5 IC2.4 IC3.4 IC4.4 IC5.4 IC8.2
DA1: IC1.4 IC2.28 IC3.28 IC4.28 IC5.28 IC8.5
DA2: IC1.3 IC2.3 IC3.3 IC4.3 IC5.3 IC8.6
DA3: IC1.2 IC2.31 IC3.31 IC4.31 IC5.31 IC8.9
DA4: IC1.1 IC2.2 IC3.2 IC4.2 IC5.2 IC8.12
DA5: IC1.48 IC2.30 IC3.30 IC4.30 IC5.30 IC8.15
DA6: IC1.17 IC2.1 IC3.1 IC4.1 IC5.1 IC8.16
DA7: IC8.19
DISK_CE_L: IC6.4 IC6.5 IC10.1 SBC.16
DX4: CF1.6 IC1.44 IC2.21 IC3.21 IC4.21 IC5.21 IC9.11
DX5: CF1.5 IC1.42 IC2.20 IC3.20 IC4.20 IC5.20 IC9.12
DX6: CF1.4 IC1.40 IC2.19 IC3.19 IC4.19 IC5.19 IC7.13 IC9.13
DX7: CF1.3 IC1.38 IC2.18 IC3.18 IC4.18 IC5.18 IC7.11 IC9.14
DX8: CF1.2 IC1.35 IC2.17 IC3.17 IC4.17 IC5.17 IC7.9 IC9.15
DX9: CF1.23 IC1.33 IC2.15 IC3.15 IC4.15 IC5.15 IC7.7 IC9.16
DX10: CF1.22 IC1.31 IC2.14 IC3.14 IC4.14 IC5.14 IC7.5 IC9.17
DX11: CF1.21 IC1.29 IC2.13 IC3.13 IC4.13 IC5.13 IC7.3 IC9.18
EMA0: IC6.3 SBC.35
EMA1: IC6.2 SBC.41
EMA2: IC6.1 SBC.21
FLASH_L: IC1.26 IC6.14
FLASH_RDY: IC1.15 IC7.6
FPGA_DONE_H: IC7.2 IC12.72
FPGA_INIT_L/RTC_CLK: IC7.4 IC12.68 IC16.7 J3.1 R3.2
FPGA_L: IC6.10 IC12.31
FPGA_PROGRAM_L: IC12.69 IC12.85 R2.2
FPGA_WR_L/RTC_IO: IC12.30 IC16.6 R7.2
G0: IC12.126 RN2.2
GND [gnd]: BATA.- BATB.- C1.- C2.- C3.2 C4.2 C5.2 C6.2 C7.2 C8.2 C9.2 C10.2 C11.2 C13.2 C14.2 C17.2 C100.2 C101.2 C102.2 C103.2 C104.2 C105.2 C106.2 C107.2 CF1.1 CF1.8 CF1.10 CF1.11 CF1.12 CF1.14 CF1.15 CF1.16 CF1.17 CF1.39 CF1.50 IC1.27 IC1.46 IC1.47 IC2.16 IC3.16 IC4.16 IC5.16 IC6.8 IC7.8 IC8.1 IC8.10 IC9.10 IC9.19 IC10.7 IC11.8 IC12.8 IC12.17 IC12.25 IC12.33 IC12.45 IC12.52 IC12.61 IC12.73 IC12.81 IC12.89 IC12.98 IC12.106 IC12.109 IC12.110 IC12.119 IC12.128 IC12.135 IC12.143 IC13.10 IC13.19 IC14.8 IC15.5 IC15.7 IC15.9 IC15.11 IC15.13 IC16.4 IC17.7 IC17.13 IO1.2 IO2.2 J3.2 JTAG.1 KBD.3 KBD.SH1 KBD.SH2 KBD.SH3 LPT.17 LPT.18 LPT.19 LPT.20 LPT.21 LPT.22 LPT.23 LPT.24 LPT.25 R4.2 R7.1 REG2.5.1 REG2.5.2 REG3.3.1 REG3.3.2 SBC.17 SBC.18 SBC.49 SER1.9 SER2.9 SER3.9 VGA.5 VGA.6 VGA.7 VGA.8 VGA.10 X1.P$2
HS: IC12.117 VGA.13
INTGNT_L: IC12.141 SBC.10
INTREQ_L: IC12.96 SBC.9
IOCLR_L: IC1.12 IC12.87 SBC.12
KB_CLK: IC12.138 KBD.6
KB_DATA: IC12.133 KBD.1
LOAD_DAR_H: IC8.11 SBC.15
LXDAR_L: IC12.18 SBC.14
MA0: IC1.6 IC2.25 IC3.25 IC4.25 IC5.25 SBC.30
MA1: IC1.7 IC2.23 IC3.23 IC4.23 IC5.23 SBC.32
MA2: IC1.8 IC2.26 IC3.26 IC4.26 IC5.26 SBC.28
MA3: IC1.18 IC2.27 IC3.27 IC4.27 IC5.27 SBC.26
MA4: IC1.19 IC2.5 IC3.5 IC4.5 IC5.5 SBC.23
MA5: IC1.20 IC2.6 IC3.6 IC4.6 IC5.6 SBC.25
MA6: IC1.21 IC2.7 IC3.7 IC4.7 IC5.7 SBC.27
MA7: IC1.22 IC2.8 IC3.8 IC4.8 IC5.8 SBC.29
MA8: IC1.23 IC2.9 IC3.9 IC4.9 IC5.9 SBC.31
MA9: CF1.18 IC1.24 IC2.10 IC3.10 IC4.10 IC5.10 SBC.33
MA10: CF1.19 IC1.25 IC2.11 IC3.11 IC4.11 IC5.11 SBC.37
MA11: CF1.20 IC1.45 IC2.12 IC3.12 IC4.12 IC5.12 SBC.39
N$1: IC12.66 IC13.2
N$2: BATA.+ R8.1
N$3: IC7.10 J3.3 R1.1
N$4: IC12.63 IC13.3
N$5: IC12.59 IC13.4
N$6: IC12.56 IC13.5
N$7: IC12.88 X1.P$3
N$8: IC16.3 X2.1
N$10: IC12.51 IC13.6
N$11: BATB.+ R11.1
N$15: IC12.43 IC13.7
N$16: IC12.47 IC13.8
N$17: IC12.38 IC13.9
N$18: IC12.28 IC13.1
N$19: IC12.7 IC15.3
N$20: IC12.10 IC15.1
N$21: IC12.137 IC17.10
N$22: IC12.91 IC17.4
N$23: IC12.121 IC17.2
N$24: IC12.136 IC17.6
N$25: IC12.124 IC17.8
N$26: IC13.18 LPT.9
N$27: IC13.17 LPT.8
N$28: IC13.16 LPT.7
N$29: IC13.15 LPT.6
N$30: IC13.14 LPT.5
N$31: IC13.13 LPT.4
N$32: IC13.12 LPT.3
N$33: IC13.11 LPT.2
N$34: IC15.2 LPT.1 R9.1
N$35: IC15.4 LPT.16 R10.1
N$36: IC17.11 LPT.15
N$37: IC17.3 LPT.10
N$38: IC17.1 LPT.11
N$39: IC17.5 LPT.12
N$40: IC17.9 LPT.13
N$41: IC12.130 IO1.26
N$42: IC12.123 IO1.24
N$43: IC12.140 IO1.22
N$44: IC12.118 IO1.20
N$45: IC12.75 IO1.18
N$46: IC12.41 IO1.16
N$47: IC12.58 IO1.14
N$48: IC12.86 IO1.12
N$49: IC12.22 IO1.10
N$50: IC12.29 IO1.8
N$51: IC12.50 IO1.6
N$52: LPT.14 R6.1
N$53: IC12.54 IO1.4
N$54: IC12.134 IO1.25
N$55: IC12.114 IO1.23
N$56: IC12.139 IO1.21
N$57: IC12.116 IO1.19
N$58: IC12.74 IO1.17
N$59: IC12.64 IO1.15
N$60: IC12.42 IO1.13
N$61: IC12.84 IO1.11
N$62: IC12.83 IO1.9
N$63: IC12.40 IO1.7
N$64: IC12.48 IO1.5
N$65: IC12.65 IO1.3
N$66: IC12.12 IO2.26
N$67: IC12.5 IO2.24
N$68: RN2.8 VGA.1
N$69: RN2.7 VGA.2
N$70: RN2.6 VGA.3
N$71: IC12.3 IO2.22
N$72: IC12.20 IO2.20
N$73: IC12.103 IO2.18
N$74: IC12.93 IO2.16
N$75: IC12.100 IO2.14
N$76: IC11.16 SER1.6
N$77: IC12.94 IO2.12
N$78: IC12.19 IO2.10
N$79: IC12.13 IO2.8
N$80: IC12.4 IO2.6
N$81: IC12.6 IO2.4
N$82: IC16.2 X2.2
N$86: CPREQ.2 IC12.113
N$91: IC9.1 IC10.3
N$92: IC11.6 IC12.23
N$93: IC11.5 IC12.11
N$94: IC11.4 IC12.26
N$95: IC11.18 IC12.21
N$96: IC11.22 IC12.27
N$97: IC11.19 IC12.115
N$101: C16.1 IC11.10
N$102: C16.2 IC11.12
N$103: C12.1 IC11.13
N$104: C12.2 IC11.14
N$105: C15.2 IC11.11
N$106: R4.1 SPKR.-
N$107: C11.1 IC11.15
N$110: IC11.7 SER2.3
N$112: IC11.3 SER3.3
N$113: IC11.24 SER1.5
N$114: IC11.23 SER1.3
R0: IC12.99 RN2.1
RAM0_L: IC6.15 IC14.4
RAM0_L_NV: IC3.22 IC14.13
RAM1_L: IC6.13 IC14.5
RAM1_L_NV: IC2.22 IC14.12
RAM2_L: IC6.11 IC14.6
RAM2_L_NV: IC5.22 IC14.11
RAM3_L: IC6.9 IC14.7
RAM3_L_NV: IC4.22 IC14.10
RD_SR_L: IC12.77 SBC.3
READ_L: CF1.9 IC1.28 IC2.24 IC3.24 IC4.24 IC5.24 IC10.2 IC12.78 SBC.11
RTC_RST: IC12.112 IC16.5
RTS2: HS2.2 IC11.21
SKIP_L: IC12.76 SBC.5
SPEAKER: IC10.6 IC10.8 IC10.11 SPKR.+
SPKR: IC10.4 IC10.5 IC10.9 IC10.10 IC10.12 IC10.13 IC12.95
STATUS_L: IC6.7 IC7.1 IC7.15
TCK: IC12.2 JTAG.4
TDI: IC12.32 JTAG.6
TDO: IC12.34 JTAG.3
TMS: IC12.142 JTAG.2
TX0: IC11.2 SER2.5
TX1: IC11.1 SER3.5
TX2: IC11.20 SER1.4
VBAT: IC14.2 IC16.8 R8.2 R11.2
VCC_NV [power]: C5.1 C6.1 C9.1 C14.1 IC2.32 IC3.32 IC4.32 IC5.32 IC14.1 IC14.3
VCCO [power2]: C2.+ C3.1 C101.1 C102.1 C104.1 C107.1 IC12.1 IC12.16 IC12.35 IC12.36 IC12.53 IC12.70 IC12.71 IC12.90 IC12.107 IC12.108 IC12.111 IC12.127 IC12.144 JTAG.5 REG2.5.3 REG2.5.4 REG3.3.5 REG3.3.6
VS: IC12.102 VGA.14
WR_SR_L: IC12.101 SBC.4
WRITE_L: CF1.36 IC1.11 IC2.29 IC3.29 IC4.29 IC5.29 IC12.15 IC12.37 SBC.13

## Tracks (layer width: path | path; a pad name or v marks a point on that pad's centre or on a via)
2V5  (via drill 0.38, 0.61)
  Top 0.254: 97.83,57.75 98.09,57.75 98.32,57.98 98.32,58.09 IC12.92 | 97.83,57.75 96.08,57.75 95.89,57.94 95.85,57.94 95.85,58.09 IC12.97 | 97.83,57.75 v97.83,57.52 97.68,57.18 v97.68,55.54 | v101.83,36.26 101.83,36.91 IC12.24 101.79,38.47 101.79,38.66 101.64,38.81 101.64,44.83 104.72,44.83 105.64,45.75 105.64,48.18 v105.79,48.53 108.92,48.53 IC12.55 | v87.05,49.25 87.24,49.06 87.69,49.06 IC12.125 89.26,49.02 89.52,49.02 89.6,48.95 v92.57,48.95 | v94.51,41.14 94.51,38.81 94.36,38.66 94.36,38.47 IC12.9 | v95.5,35.8 96.8,35.8 96.8,36.91 IC12.14 | v103.16,55.54 103.16,57.75 103.31,57.9 103.31,58.09 IC12.82 | v110.06,57.75 109.52,58.28 109.32,58.49
  Top 0.61: v106.25,81.97 106.22,81.94 | v110.31,61.24 110.31,59.49 109.32,58.49 v105.41,54.58 | 106.22,81.94 REG2.5.5 | 106.22,81.94 106.22,83.21 REG2.5.6 | C1.+ 105.59,91.87 v108.51,91.87
  Route2 0.254: v95.5,35.8 95.5,38.13 94.67,38.96 94.67,40.79 v94.51,41.14
  Route2 0.61: v108.51,91.87 108.51,83.77 106.22,81.94 v106.25,81.97
  Bottom 0.254: v97.83,57.52 97.83,60.83 C105.1 | v101.83,36.26 100.99,35.42 100.04,35.42 C100.1 | v87.05,49.25 86.7,49.59 86.7,49.75 C103.1 | v94.51,41.14 94.51,41.81 | 105.41,48.53 v105.79,48.53 | 103.16,54.66 v103.16,55.54 | v110.06,57.75 112.69,55.12 112.69,51.04 C106.1 | 92.89,48.95 v92.57,48.95 | 97.68,54.66 v97.68,55.54
  Bottom 0.61: v106.25,81.97 106.25,65.66 108.74,62.92 109.19,62.41 v110.31,61.24
  Bottom 0.813: v105.41,54.58 105.41,48.53 105.41,41.81 94.51,41.81 92.89,41.81 92.89,48.95 92.89,54.66 97.68,54.66 103.16,54.66 105.54,54.66
5V  (via drill 0.38)
  Top 0.254: 11.57,97.26 11.34,97.26 IC1.14 | v12.29,77.47 12.22,77.44 12.22,78.05 IC1.37 | v12.24,75.95 10.73,74.43 C8.1 | v11.61,96.65 11.61,97.14 11.57,97.26 | v26.12,70.4 26.12,69.79 26.12,69.67 IC10.14 28.11,69.18 30.2,69.18 C13.1 | v23.88,22.62 24.49,22.62 CF1.44 | v23.11,29.97 23.23,30.09 24.49,30.09 CF1.38 24.49,30.35 24.49,30.62 CF1.13 26.43,30.85 27.76,30.85 27.76,36.56 | v30.43,46.09 31.04,46.09 R5.2 | 137.53,26.35 137.53,28.45 R10.2 137.49,29.97 137.07,30.39 134.06,30.39 133.68,30.01 R9.2 | 137.53,26.35 137.53,25.74 IC15.14 | 136.14,16.15 135.97,16.33 122.94,16.33 121.6,15 IC16.1 121.03,12.87 114.9,12.87 113.79,11.76 IO2.1 | 136.14,16.15 136.73,15.57 IC17.14 | v137.41,26.35 137.53,26.35 | v136.84,16.85 136.14,16.15 | v146.76,68.29 146.06,68.99 136.16,68.99 C10.1 134.71,69.63 130.48,73.86 130.48,76.61 122.06,76.61 117.03,71.58 116.46,71.58 115.13,72.91 115.13,76.95 114.67,76.95 114.25,77.37 R1.2 112.99,77.44 | 139.95,43.54 141.49,43.54 R6.2 143.01,44.79 143.01,55.35 149.64,61.98 KBD.5 | 139.95,43.54 139.4,43.54 IC13.20 137.41,44.15 132.69,48.87 132.69,51.19 C15.1 131.17,52.95 125.49,58.62 123.28,58.62 IC11.9 | 139.95,43.54 v139.95,41.94 | REG3.3.3 112.8,83.22 | 110.53,77.41 110.45,77.32 110.36,77.41 C7.1 | 111.13,81.67 REG3.3.4 | v25.18,71.46 26.44,72.72 26.43,72.69 26.57,72.83 38.24,72.86 38.38,72.72 38.39,72.72 39.08,72.03 44.87,72.03 44.87,71.92 IC8.20 46.85,72.03 62.09,72.03 62.43,71.69 IC9.20 64.41,71.08 67.31,71.08 67.31,70.24 70.82,66.74 SBC.1 | 111.16,77.44 110.97,77.41 C7.1 | X1.P$1 108.5,69.75 108.5,72.26 X1.P$4 108.5,74.02 v107.89,74.02
  Top 0.254: v101.1,61.48 99.43,61.48 98.29,62.62 R2.1 | 102.13,75.73 IC7.16 | v107.89,75.43 107.89,75.92 107.89,76.04 | 111.13,78.89 111.05,78.7 C7.1 | v92.19,64.72 92.19,64.11 R3.1 | 86.22,75.58 IC6.16 | 94.59,78.55 v94.97,78.7 | IC6.6 80,68.64 77.75,66.4 74.36,66.4 SBC.2 | 62.62,34.85 62.05,35.42 C17.1 60.8,36.91 60.8,38.2 29.48,38.2 27.88,36.6 27.76,36.56 | 62.62,34.85 62.66,34.85 | 27.76,36.56 26.62,37.71 26.43,37.71 CF1.32 | IC14.16 62.66,34.73 62.62,34.85 | 11.57,97.26 IC1.13
  Top 0.406: REG3.3.4 110.4,81.93 110.4,83.21 REG3.3.3 | 112.8,83.22 114.78,83.22 114.78,86.54 C4.1 | 110.45,77.32 109.16,76.04 107.89,76.04 104.04,76.04 103.63,75.43 IC7.16 | 111.16,77.44 112.99,77.44 | 111.13,78.89 111.13,81.67 | v102.13,77.1 102.13,75.73 | 86.22,75.96 86.22,77.55 87.36,77.55 88.37,78.55 94.59,78.55 | 86.22,75.96 86.22,75.58 | v76.3,73.98 76.57,73.98 78.65,76.06 86.03,76.06 86.22,75.96
  Route2 0.406: v94.97,78.7 95.85,77.83 99.05,77.83 99.62,77.25 101.75,77.25 v102.13,77.1
  Route2 0.61: SBC.1 SBC.2
  Bottom 0.254: v12.24,75.95 12.22,77.37 v12.29,77.47 12.56,77.67 12.56,85.18 | v11.61,96.65 12.56,95.69 12.56,85.18 | 25.13,71.39 23,73.52 23,82.27 20.12,85.18 12.56,85.18 | 25.13,71.39 v26.12,70.4 26.28,70.05 31.04,65.29 31.04,61.67 33.9,58.81 33.9,49.75 30.58,46.43 v30.43,46.09 23.11,38.77 v23.11,29.97 23.11,23.38 v23.88,22.62 | IO1.1 113.37,23.42 114.17,22.62 114.17,12.98 113.37,12.18 IO2.1 | v136.84,16.85 136.84,25.78 v137.41,26.35 137.57,26.7 139.93,29.06 v139.95,41.94 | v146.76,68.29 148.88,66.17 148.88,64.11 149.64,63.35 KBD.5 | 25.13,71.39 v25.18,71.46 | v101.1,61.48 102.48,62.85 102.48,75.77 102.13,76.11 v102.13,77.1 | v107.89,75.43 v107.89,74.02 | v94.97,78.7 93.31,76.88 93.31,74.41 93.69,74.03 93.7,71.63 93.67,71.6 93.67,71.57 93.33,71.23 93.29,71.2 92.53,70.43 92.53,65.06 v92.19,64.72
  Bottom 0.406: v76.3,73.98 74.02,71.69 74.02,66.74 SBC.2
B0  (via drill 0.38)
  Top 0.178: v89.87,51.61 89.26,51.61 IC12.120 | v89.1,65.94 90.13,66.97 90.97,66.97 92.49,68.49 96.77,68.49 98.41,70.97 104.01,70.97 107.62,74.74 110.63,74.74 118.25,67.12 129.18,67.12 130.48,65.82 141.11,65.82 141.87,65.06 RN2.3
  Bottom 0.178: v89.87,51.61 88.84,52.64 88.84,60.38 89.1,60.64 v89.1,65.94
C0_L  (via drill 0.38)
  Top 0.178: v104.99,57.52 104.91,57.52 104.91,58.09 IC12.79
  Route2 0.178: v102.98,76.4 99.75,76.4 99.2,76.95 92.72,76.95 85.41,69.63 83.58,69.63 74.66,60.72 74.66,60.53 73.73,59.59 72.7,59.59 71.84,58.74 SBC.7
  Bottom 0.178: v104.99,57.52 103.09,59.42 103.09,62.28 102.9,62.47 102.9,76.34 v102.98,76.4
C1_L  (via drill 0.38)
  Top 0.178: v104.5,60.49 104.38,60.49 104.38,59.65 IC12.80 | v103.54,65.56 103.2,65.9 96.65,65.9 96.61,65.94 93.56,65.94 93.1,65.48 90.53,65.48 86.89,61.82 v76.68,61.82
  Bottom 0.178: v104.5,60.49 104.38,60.6 104.38,64.72 v103.54,65.56 | v76.68,61.82 74.02,59.16 74.02,59.12 SBC.8
CF_DETECT_L  (via drill 0.38)
  Top 0.178: CF1.26 26.43,45.4 31.04,45.4 R5.1 32.52,45.48 34.39,47.35 56.18,47.35 v56.79,47.96 | v98.51,69.82 100.5,69.82 100.77,70.09 IC7.12 | v97.87,76.07 96.99,76.95 92.74,76.95 92.43,76.64 v89.6,76.64
  Route2 0.178: v89.6,76.64 88.28,76.64 73.61,62.03 73.53,62.03 70.86,62.03 70.75,62.03 70.7,61.98 56.79,48.07 v56.79,47.96
  Bottom 0.178: v98.51,69.82 97.87,70.47 v97.87,76.07
CF_L  (via drill 0.38)
  Top 0.178: v79.77,48.18 78.52,46.94 69.24,46.94 68.3,47.88 62.74,47.88 61.48,46.62 36.87,46.62 28.83,38.58 26.43,38.58 CF1.7 | v84.57,68.72 85.75,69.9 86.17,69.9 IC6.12
  Bottom 0.178: v79.77,48.18 80.45,48.87 80.45,60.34 84.26,64.15 84.26,68.41 v84.57,68.72
CF_READY  (via drill 0.38)
  Top 0.178: v27,31.57 26.43,31.57 CF1.37 | v47.84,54.85 50.43,57.44 82.13,57.44 v83.08,58.39 | 94.37,74.87 v94.05,74.8 94.36,74.86 | 94.36,74.86 | 94.36,74.86 | 94.36,74.86 | 94.36,74.86 99.03,74.86 | 99.03,74.86 99.02,74.87 99.03,74.86 | 99.03,74.86 100.94,72.97 IC7.14 | 94.36,74.86 | 94.36,74.86 | 94.36,74.86
  Route2 0.178: v83.08,58.39 83.46,58.39 86.51,61.44 88.46,61.44 v89.75,62.74
  Bottom 0.178: v27,31.57 37.9,42.47 37.9,44.91 v47.84,54.85 | v89.75,62.74 91.05,64.03 94.78,64.03 94.78,74.15 v94.05,74.8
CPUDX0  (via drill 0.38)
  Top 0.178: v82.28,47.42 85.33,50.47 87.69,50.47 IC12.122 | v80.42,25.63 80.23,25.44 74.36,25.44 SBC.34 | v105.26,6.85 104.99,7.11 v90.82,7.11
  Bottom 0.178: v82.28,47.42 81.94,47.08 81.94,27.15 v80.42,25.63 80.57,25.29 80.57,19.04 83.62,15.99 83.62,7.11 v90.82,7.11 | v105.26,6.85 107.39,6.85 109.03,8.48 109.03,9.59 110.17,10.73 IO2.3
CPUDX1  (via drill 0.38)
  Top 0.178: v89.87,45.48 89.26,45.48 IC12.132 | v94.67,20.37 94.48,20.56 89.48,20.56 v89.14,20.71 88.99,20.56 76.38,20.56 74.36,22.58 SBC.36
  Route2 0.178: v94.67,20.37 96.53,20.37 100.08,16.83 102.78,16.83 107.54,12.07 IO2.5
  Bottom 0.178: v89.87,45.48 89.37,44.98 89.37,28.26 89.64,27.99 89.64,25.1 89.14,24.6 v89.14,20.71
CPUDX2  (via drill 0.38)
  Top 0.178: v94.51,46.74 89.75,46.74 89.52,46.96 89.26,46.96 IC12.129 | v80.38,30.96 76.15,26.73 73.56,26.73 72.68,25.86 72.68,21.02 73.37,21.02 SBC.38 74.36,20.03 76.04,18.35 98.55,18.35 100.08,16.83 v105.37,16.83
  Route2 0.178: v94.51,46.74 94.51,45.1 87.69,38.28 87.69,37.9 80.76,30.96 v80.38,30.96
  Bottom 0.178: v105.37,16.83 105.37,12.18 IO2.7
CPUDX3  (via drill 0.38)
  Top 0.178: v93.87,45.78 93.52,46.13 89.6,46.13 89.56,46.09 89.26,46.09 IC12.131 | v87.05,31.38 81.94,26.28 75.46,26.28 v75.27,26.09 | v98.59,17.4 98.17,17.82 74.36,17.82 SBC.40
  Route2 0.178: v93.87,45.78 93.87,44.98 v87.05,38.16 | v98.59,17.4 102.55,13.44 102.55,12.18 IO2.9
  Bottom 0.178: v87.05,31.38 v87.05,38.16 | v75.27,26.09 75.16,25.81 75.16,19.69 73.98,18.5 SBC.40
CPUDX4  (via drill 0.38)
  Top 0.178: v111.05,54.17 110.74,54.47 110.48,54.47 IC12.67 | v98.59,15.04 97.71,15.91 74.7,15.91 74.36,15.57 SBC.42 72.99,15.57 72.3,16.26 72.29,16.27 72.13,16.28 65.66,16.28 v65.56,16.18 | 55.58,61.52 55.58,68.34 54.51,69.41 46.85,69.41 IC8.18 | 55.58,61.52 54.36,61.52 IC9.9 | v55.92,61.14 55.61,61.44 55.58,61.52
  Bottom 0.178: v111.05,54.17 110.02,53.14 110.02,35.19 109.03,34.2 109.03,14.01 106.48,11.46 106.48,11 105.45,9.97 104.04,9.97 104.04,8.56 103.35,7.87 101.41,7.87 101.41,10.01 100.69,10.73 IO2.11 99.96,12.1 98.59,13.47 v98.59,15.04 | v55.92,61.14 57.63,59.42 57.63,24.1 v65.56,16.18
CPUDX5  (via drill 0.38)
  Top 0.178: v49.67,68.31 49.5,68.15 49.02,68.15 46.85,68.15 IC8.17 | v51.8,62.59 52.37,62.59 IC9.8 | v111.05,51.96 110.48,51.96 IC12.62 | v110.71,13.06 110.13,12.48 99.28,12.48 98.55,11.76 IO2.13 | v52.37,23.04 62.36,13.06 70.47,13.06 SBC.43
  Bottom 0.178: v49.67,68.31 51.8,66.01 v51.8,62.59 51.96,62.24 52.37,61.82 v52.37,23.04 | v111.05,51.96 110.78,51.69 110.78,35.12 111.54,34.35 111.54,13.89 v110.71,13.06 | IO2.13 97.49,10.73 96.76,10.01 96.76,4.94 76.64,4.94 76.15,5.44 75.32,6.25 73.66,6.25 72.68,7.23 72.68,10.77 71.42,12.03 SBC.43
CPUDX6  (via drill 0.38)
  Top 0.178: 51.08,63.84 52.37,63.84 IC9.7 | 51.08,63.84 50.93,63.69 50.86,63.69 47.03,63.69 47,63.69 46.85,63.84 IC8.14 | v103.16,47.73 105.3,49.86 107.51,49.86 108.61,50.97 108.92,50.97 IC12.60 | v80.11,11.19 74.86,11.19 72.69,11.19 72.57,11.19 71.84,10.46 SBC.45 70.47,10.5 63.61,10.5 v51.08,23.04 | v51.08,63.77 51.08,63.84
  Route2 0.178: v103.16,47.73 103.16,44.45 99.35,40.64 99.35,34.81 v96.8,32.18
  Bottom 0.178: v96.8,32.18 96.38,31.65 96.38,13.28 95.62,12.52 95.62,12.18 IO2.15 94.93,10.73 94.25,10.05 94.25,5.7 84.3,5.7 81.52,8.48 81.52,9.78 v80.11,11.19 | v51.08,23.04 v51.08,63.77
CPUDX7  (via drill 0.38)
  Top 0.178: 50.43,63.12 51.42,63.12 51.54,63.23 52.15,63.23 52.22,63.16 54.51,63.16 54.66,63.31 54.66,64.72 54.36,64.72 IC9.6 | 50.43,63.12 46.85,63.12 IC8.13 | v102.51,46.16 105.83,49.48 108.92,49.48 IC12.57 | v84.57,6.35 72.83,6.35 71.84,7.34 SBC.47 | v50.43,62.81 50.43,63.12
  Route2 0.178: v102.51,46.16 102.51,44.34 98.97,40.79 98.97,38.35 v93.83,33.21
  Bottom 0.178: v93.83,33.21 93.83,12.94 93.07,12.18 IO2.17 92.42,10.73 91.69,10.01 91.69,6.35 v84.57,6.35 | v50.43,62.81 50.43,22.77 68.41,4.79 70,4.79 70.17,6.27 70.85,6.96 SBC.47
CPUDX8  (via drill 0.38)
  Top 0.178: IC8.8 36.79,63.16 37.52,63.88 44.07,63.88 44.56,64.38 44.56,64.76 48.02,64.76 48.54,64.24 48.59,64.17 48.69,64.17 50.53,64.17 50.57,64.17 50.66,64.26 52.37,65.98 IC9.5 54.36,65.98 54.66,65.67 v54.93,65.67 | v108.31,45.9 108.61,45.59 108.92,45.59 IC12.49 | v112,54.81 112.65,54.17 116.5,54.17 v118.44,52.22 | v115.32,9.66 113.14,7.49 97.75,7.49 96.3,8.94 96.3,10.43 91.66,10.43 90.93,11.15 IO2.19 89.45,11.15 88.57,10.27 86.63,10.27 86.63,8.94 85.18,7.49 75.73,7.49 v75.23,7 | v66.89,7.99 68.72,6.13 72.23,6.13 72.99,5.4 SBC.50
  Route2 0.178: v75.23,7 74.02,5.78 SBC.50
  Bottom 0.178: v108.31,45.9 109.64,47.23 109.64,53.67 110.78,54.81 v112,54.81 | v118.44,52.22 119.77,50.89 119.77,27.84 119.93,27.69 119.93,18.92 115.32,14.31 v115.32,9.66 | v54.93,65.67 55.27,65.33 55.27,19.61 v66.89,7.99
CPUDX9  (via drill 0.38)
  Top 0.178: v43.8,64.53 36.87,64.53 36.79,64.45 IC8.7 | v50.91,65.43 52.07,66.59 52.07,67.27 52.37,67.27 IC9.4 | v111.43,43.19 110.67,43.95 110.48,43.95 IC12.46 | v111.93,13.36 111.58,13.7 101.33,13.7 100.65,14.39 v90.36,14.39 | IO2.21 86.93,11.11 86.13,10.31 84.07,10.31 84.07,8.9 83.05,7.87 74.36,7.87 SBC.48 72.99,7.95 72.3,8.64 72.25,8.69 72.19,8.69 62.69,8.69 62.56,8.71 62.57,8.71 v49.78,21.48
  Bottom 0.178: 49.78,64.53 50.91,64.53 v50.91,65.43 | 49.78,64.53 v43.8,64.53 | v111.43,43.19 111.54,43.08 111.54,34.89 111.93,34.51 v111.93,13.36 | v90.36,14.39 88.07,12.1 IO2.21 | v49.78,21.48 49.78,64.53
CPUDX10  (via drill 0.38)
  Top 0.178: 43.27,68.61 48.94,68.61 49.13,68.8 49.19,68.86 49.2,68.86 49.36,69.03 50.03,69.03 50.27,68.78 50.29,68.78 52.37,68.8 IC9.3 | 43.27,68.61 37.13,68.61 36.79,68.26 IC8.4 | v104.46,42.77 108.42,42.77 108.61,42.96 108.92,42.96 IC12.44 | v85.56,13.74 v99.24,13.74 | IO2.23 84.38,11.15 83.65,10.43 74.36,10.43 SBC.46 72.99,9.89 72.3,9.21 72.21,9.21 72.19,9.19 63.03,9.19 63.01,9.21 62.97,9.21 v49.14,23.04 | v43.27,68.53 43.27,68.61
  Route2 0.178: v104.46,42.77 104.46,42.13 101.18,38.85 101.18,35.76 v101.83,35.12
  Bottom 0.178: v101.83,35.12 100.34,33.63 100.34,25.63 99.24,24.52 v99.24,13.74 | v85.56,13.74 85.45,13.63 85.45,12.18 IO2.23 | v43.27,68.53 43.15,68.41 43.15,60.45 48.49,55.12 48.49,23.69 v49.14,23.04
CPUDX11  (via drill 0.38)
  Top 0.178: IC8.3 36.79,69.52 37.1,69.82 52.37,69.82 IC9.2 54.36,69.82 v55,69.82 | v108.31,39.99 108.8,40.49 108.92,40.49 IC12.39 | v106.67,25.25 106.67,20.1 95.31,20.1 94.93,19.72 90.7,19.72 v90.59,19.84 | v86.86,14.92 86.32,14.39 85.26,14.39 82.97,12.1 IO2.25 81.9,11.84 74.93,11.84 74.36,12.41 SBC.44 72.99,13.02 72.25,13.75 69.16,13.75 v67.31,15.61
  Bottom 0.178: v108.31,39.99 108,39.69 108,28.45 106.67,27.11 v106.67,25.25 | v90.59,19.84 86.86,16.1 v86.86,14.92 | v55,69.82 55.65,69.18 55.65,62.32 57.98,59.99 57.98,31.99 59.35,30.62 60.74,30.62 60.87,30.73 61.25,31.12 63.27,31.12 63.27,19.65 v67.31,15.61
CTS2
  Top 0.178: IC11.17 133.34,60.41 134.52,61.6 139.2,61.6 HS2.1
DA0  (via drill 0.38)
  Top 0.178: v18.48,99.12 15.76,99.12 15.76,98.82 IC1.5 | v22.06,95.54 22.71,94.89 25.55,94.89 IC2.4 27.72,94.89 29.25,96.42 36.94,96.42 v37.21,96.15 | v43.27,70.47 36.79,70.47 IC8.2 | v43.31,94.59 44.6,94.59 IC3.4 46.77,94.36 47,94.36 47.31,94.06 59.69,94.06 59.96,94.32 63.58,94.32 63.65,94.4 IC4.4 65.82,94.36 66.05,94.36 66.36,94.06 78.74,94.06 79.01,94.32 83.96,94.32 84,94.36 IC5.4
  Route2 0.178: v37.21,96.15 40.41,96.15 41.82,94.74 42.96,94.74 v43.31,94.59
  Bottom 0.178: v22.06,95.54 v18.48,99.12 | v43.27,70.47 43.31,70.51 v43.31,94.59
DA1  (via drill 0.38)
  Top 0.178: v17.25,95.54 16.26,95.54 16.26,97.26 IC1.4 | v29.17,94.7 30.24,93.64 38.35,93.64 IC2.28 40.53,93.64 40.83,93.94 46.89,93.94 47.16,93.68 57.37,93.68 57.4,93.64 IC3.28 59.58,93.64 59.8,93.64 60.11,93.94 65.94,93.94 66.21,93.68 76.42,93.68 76.45,93.64 IC4.28 78.63,93.64 78.85,93.64 79.16,93.94 96.49,93.94 96.8,93.64 IC5.28 | v30.81,68.22 33.56,68.22 34.81,66.97 IC8.5
  Bottom 0.178: v17.25,95.54 18.2,94.59 27.57,94.59 | 27.57,94.59 27.84,94.59 27.95,94.7 v29.17,94.7 | v30.81,68.22 27.57,71.44 27.57,94.59
DA2  (via drill 0.38)
  Top 0.178: v37.4,65.67 36.79,65.67 IC8.6 | IC5.3 84,95.81 79.24,95.81 78.74,95.31 66.4,95.31 66.05,95.66 65.82,95.66 IC4.3 63.65,95.66 63.61,95.62 61.67,95.62 61.37,95.31 47.35,95.31 47,95.66 46.77,95.66 IC3.3 44.6,95.89 v41.59,95.89 41.25,96.04 41.1,96.04 40.64,96.49 38.35,96.49 38.05,96.8 29.1,96.8 28.52,96.23 27.76,96.23 27.72,96.19 IC2.3 25.59,96.19 16.75,96.19 16.75,97.26 IC1.3
  Bottom 0.178: v37.4,65.67 41.59,69.86 v41.59,95.89
DA3  (via drill 0.38)
  Top 0.178: IC5.31 96.8,97.45 96.49,97.75 78.93,97.75 78.63,97.45 IC4.31 76.45,97.45 76.34,97.56 v75.88,97.56 | 31.46,97.18 28.68,97.18 28.11,96.61 17.28,96.61 17.28,97.26 IC1.2 | 31.46,97.18 IC2.31 40.53,96.91 40.75,96.91 41.14,96.53 46.81,96.53 47.46,97.18 IC3.31 59.58,97.1 v61.71,97.1 | v34.24,62.47 34.81,61.9 IC8.9 | v31.46,97.45 31.46,97.18
  Bottom 0.178: v34.24,62.47 31.46,65.25 v31.46,97.45 | v75.88,97.56 61.71,97.56 v61.71,97.1
DA4  (via drill 0.38)
  Top 0.178: v42.51,63.23 43.54,63.23 44.87,61.9 IC8.12 | v43.23,97.18 IC3.2 46.77,97.45 46.89,97.56 47.7,97.56 47.89,97.75 63.35,97.75 63.65,97.45 IC4.2 65.82,96.91 75.73,96.91 76.04,96.61 83.69,96.61 84,96.91 IC5.2 | v28.37,97.79 28.07,97.79 27.72,97.45 IC2.2 25.55,97.26 17.82,97.26 IC1.1
  Route2 0.178: v28.37,97.79 30.89,97.79 31.19,98.09 42.13,98.09 42.89,97.33 v43.23,97.18
  Bottom 0.178: v42.51,63.23 42.62,63.35 42.62,96.57 v43.23,97.18
DA5  (via drill 0.38)
  Top 0.178: 75.94,96.17 75.96,96.15 76.45,96.15 IC4.30 | 75.94,96.17 75.62,96.49 62.01,96.49 61.44,95.92 59.58,95.92 IC3.30 57.4,96.15 57.02,96.53 v55.99,96.53 | v96.19,95.96 96.8,95.96 IC5.30 | v75.88,95.96 75.88,96.11 75.94,96.17 | v32.11,77.94 17.93,77.94 17.82,78.05 IC1.48 | v37.44,67.96 39.69,65.71 44.87,65.71 IC8.15 | v37.91,95.28 37.97,95.28 38.35,95.66 IC2.30
  Bottom 0.178: v75.88,95.96 v96.19,95.96 | v37.44,67.96 37.44,72.61 v32.11,77.94 32.26,78.28 33.06,79.08 33.06,90.4 v37.91,95.28 38.09,95.52 38.09,99.39 53.14,99.39 v55.99,96.53
DA6  (via drill 0.38)
  Top 0.178: v9.78,99.39 9.78,98.82 IC1.17 | v18.43,97.98 18.66,98.21 25.55,98.21 IC2.1 27.72,98.44 37.59,98.44 38.2,99.05 42.05,99.05 v42.24,98.74 42.28,98.7 44.6,98.7 IC3.1 46.77,98.7 47.12,99.05 59.73,99.05 60.34,98.44 63.65,98.44 IC4.1 65.82,98.7 66.24,99.12 83.62,99.12 84,98.74 IC5.1 | v41.97,67.88 43.95,67.88 44.87,66.97 IC8.16
  Bottom 0.178: v9.78,99.39 11.19,97.98 v18.43,97.98 | v41.97,67.88 42.24,68.15 v42.24,98.74
DISK_CE_L  (via drill 0.38)
  Top 0.178: v22.92,69.18 21.97,69.18 IC10.1 | v33.17,53.56 36.87,49.86 70.7,49.86 71.27,49.29 72.26,49.29 72.99,48.56 SBC.16 74.36,48.6 75.12,48.6 v75.5,48.98 | IC6.4 80,71.16 80,70.51 IC6.5 80,70.17 v78.36,70.17
  Bottom 0.178: v22.92,69.18 33.17,58.93 v33.17,53.56 | v78.36,70.17 78.05,69.86 78.05,51.54 v75.5,48.98
DX4  (via drill 0.38)
  Top 0.178: v57.71,64.38 60.99,61.1 61.6,61.1 62.43,60.26 IC9.11 | IC5.21 96.8,84.49 86.86,84.49 86.28,85.06 79.2,85.06 78.85,84.72 78.63,84.72 IC4.21 76.45,84.72 66.28,84.72 65.94,85.06 60.57,85.06 60.26,84.76 59.58,84.76 IC3.21 57.4,84.49 v56.83,84.49 56.49,84.65 56.03,85.1 41.55,85.1 41.17,84.72 40.53,84.72 IC2.21 38.35,84.72 37.02,84.72 36.64,85.1 18.39,85.1 v17.13,83.85 | v15.68,77.44 15.68,78.05 IC1.44 | v18.47,45.71 24.33,39.84 24.49,39.84 CF1.6
  Bottom 0.178: v57.71,64.38 57.21,64.87 57.21,84.11 v56.83,84.49 | 15.04,76.8 v15.68,77.44 | 15.04,76.8 13.89,76.8 13.89,79.39 14.54,80.04 14.54,81.25 v17.13,83.85 | v18.47,45.71 15.08,49.1 15.08,76.72 15.04,76.8
DX5  (via drill 0.38)
  Top 0.178: v56.57,66.43 61.52,61.48 62.43,61.48 IC9.12 | IC5.20 96.8,83.5 96.49,83.81 79.65,83.81 79.31,83.46 78.63,83.46 IC4.20 76.45,83.46 76.42,83.5 66.24,83.5 65.94,83.81 61.14,83.81 60.8,83.46 59.58,83.46 IC3.20 57.4,83.35 v56.57,83.35 56.22,83.5 55.92,83.81 41.1,83.81 40.75,83.46 40.53,83.46 IC2.20 38.35,83.46 28.18,83.46 27.84,83.81 18.31,83.81 v18.28,83.85 | v14.54,77.44 14.66,77.44 14.66,78.05 IC1.42 | v18.47,47 24.37,41.1 24.49,41.1 CF1.5
  Bottom 0.178: v56.57,83.35 v56.57,66.43 | v14.54,77.44 14.92,77.83 14.92,79.04 | 14.92,79.04 14.92,80.49 v18.28,83.85 | v18.47,47 16.33,49.14 16.33,77.71 15,79.04 14.92,79.04
DX6  (via drill 0.38)
  Top 0.178: v68.91,67.27 64.41,62.78 IC9.13 62.43,62.17 62.4,62.13 v61.79,62.13 | v69.22,82.02 76.45,82.02 IC4.19 78.63,82.21 78.85,82.21 79.16,82.51 96.49,82.51 96.8,82.21 IC5.19 98.03,81.86 98.86,81.86 v103.69,77.03 | v13.78,80.19 13.78,79.62 IC1.40 | v14.16,82.47 14.24,82.55 v20.03,82.55 37.59,82.55 37.94,82.21 38.35,82.21 IC2.19 40.53,82.21 40.75,82.21 41.06,82.51 46.89,82.51 47.16,82.25 57.37,82.25 57.4,82.21 IC3.19 | v18.47,48.26 24.33,42.39 24.49,42.39 CF1.4 26.43,42.39 31.24,42.39 35.82,46.96 59.65,46.96 v60.64,47.96 | v103.69,71.69 102.86,71.69 102.36,71.69 101.69,71.69 IC7.13
  Bottom 0.178: v68.91,67.27 69.22,67.58 v69.22,82.02 | v13.78,80.19 14.16,80.57 v14.16,82.47 | v18.47,48.26 17.82,48.91 17.82,81.56 18.81,82.55 v20.03,82.55 | v61.79,62.13 60.64,60.99 v60.64,47.96 | v103.69,77.03 v103.69,71.69
DX7  (via drill 0.38)
  Top 0.178: v61.79,71.23 61.14,71.23 61.14,65.37 62.43,64.07 IC9.14 | v99.96,69.18 101.1,69.18 IC7.11 | v99.81,78.54 99.81,80.26 99.05,80.26 98.93,80.38 IC5.18 96.8,80.68 86.86,80.68 86.28,81.25 79.2,81.25 78.89,80.95 78.63,80.95 IC4.18 76.45,80.91 76.38,80.99 66.21,80.99 65.94,81.25 61.82,81.25 61.25,80.68 v60.91,80.53 59.58,80.53 IC3.18 57.4,80.91 57.33,80.99 47.16,80.99 46.89,81.25 41.1,81.25 40.79,80.95 40.53,80.95 IC2.18 38.35,80.91 37.94,80.91 37.59,81.25 20.56,81.25 | 20.56,81.25 12.75,81.25 12.75,79.62 IC1.38 | v23.3,44.68 24.33,43.65 24.49,43.65 CF1.3 | v20.56,81.06 20.56,81.25
  Bottom 0.178: v61.79,71.23 61.79,79.65 v60.91,80.53 | v99.96,69.18 99.77,69.53 99.77,75.77 99.81,75.81 v99.81,78.54 | v23.3,44.68 20.56,47.42 v20.56,81.06
DX8  (via drill 0.38)
  Top 0.178: v61.79,65.98 62.43,65.33 IC9.15 | 60.49,78.74 60.49,79.12 59.58,79.12 IC3.17 57.4,79.16 56.98,78.74 40.91,78.74 40.53,79.12 IC2.17 38.35,79.16 37.94,78.74 22.28,78.74 | 60.49,78.74 v60.49,77.06 | 60.49,78.74 65.86,78.74 66.01,78.89 76.19,78.89 76.45,79.16 IC4.17 78.63,79.65 78.85,79.65 79.24,80.04 83.62,80.04 83.65,80 86.25,80 86.86,79.39 96.8,79.39 IC5.17 98.93,79.12 99.16,79.12 v99.16,76.07 | v99.16,66.55 IC7.9 | v11.15,77.44 11.15,78.05 IC1.35 | v19.27,78.59 19.42,78.74 22.28,78.74 | v27,44.75 26.43,44.75 CF1.2 | v22.28,78.59 22.28,78.74
  Route2 0.178: v11.15,77.44 11.34,77.5 12.43,78.59 v19.27,78.59
  Bottom 0.178: v61.79,65.98 60.49,67.27 v60.49,77.06 | v99.16,76.07 v99.16,66.55 | v27,44.75 27,64.19 22.28,68.91 v22.28,78.59
DX9  (via drill 0.38)
  Top 0.178: v61.79,67.23 62.43,66.59 IC9.16 | v97.16,67.94 96.08,67.94 IC7.7 | v96.32,80.04 96.05,80.3 86.47,80.3 86.4,80.38 86.13,80.38 IC5.15 84,80.42 79.08,80.42 78.74,80.07 66.17,80.07 65.82,80.42 IC4.15 63.65,80.42 62.17,80.42 v61.14,79.39 60.8,79.54 60.34,80 47.19,80 46.77,80.42 IC3.15 44.6,80.42 44.26,80.07 28.07,80.07 27.72,80.42 IC2.15 25.55,80.42 19.34,80.42 v18.47,79.54 | v11.84,80.19 10.27,80.19 10.27,79.62 IC1.33 | v23.88,18.24 24.49,18.24 CF1.23
  Route2 0.178: v11.84,80.19 12.87,80.19 13.51,79.54 v18.47,79.54
  Bottom 0.178: v61.79,67.23 61.14,67.88 v61.14,79.39 | v97.16,67.94 97.22,68.34 97.22,79.16 v96.32,80.04 | v23.88,18.24 19.11,23 19.11,61.18 18.62,61.67 18.62,79.2 v18.47,79.54
DX10  (via drill 0.38)
  Top 0.178: v66.59,70.05 64.41,67.88 IC9.17 | v87.12,81.33 86.78,81.67 86.13,81.67 IC5.14 84,81.67 83.96,81.64 79.04,81.64 78.78,81.37 67.2,81.37 v66.97,81.64 66.93,81.67 65.82,81.67 IC4.14 63.65,81.67 61.71,81.67 61.4,81.37 57.29,81.37 57.02,81.64 46.81,81.64 46.77,81.67 IC3.14 44.6,81.67 44.56,81.64 40.94,81.64 40.68,81.37 38.01,81.37 37.71,81.67 27.72,81.67 IC2.14 25.55,81.83 19.08,81.83 | v91.39,70.36 IC7.5 | 19.08,81.83 9.28,81.83 9.28,79.62 IC1.31 | v23.88,19.53 24.49,19.53 CF1.22 | v19.08,81.9 19.08,81.83
  Bottom 0.178: v66.59,70.05 66.97,70.43 v66.97,81.64 | v91.39,70.36 91.39,77.06 v87.12,81.33 | v23.88,19.53 19.99,23.42 19.99,79.04 18.69,80.34 18.69,81.52 v19.08,81.9
DX11  (via drill 0.38)
  Top 0.178: v65.44,70.17 64.41,69.14 IC9.18 | 83.39,82.89 79.01,82.89 78.74,82.63 70.17,82.63 70.13,82.66 66.62,82.66 v66.28,82.6 65.9,82.93 65.82,82.93 IC4.13 63.65,82.97 63.31,82.63 56.38,82.63 56.11,82.89 46.81,82.89 46.77,82.93 IC3.13 44.6,82.97 44.53,82.89 40.91,82.89 40.64,82.63 38.05,82.63 37.74,82.93 27.72,82.93 IC2.13 25.55,83.2 9.25,83.2 v7.42,81.37 | 83.39,82.89 83.96,82.89 84,82.93 IC5.13 | v92.83,73.79 92.83,73.55 93.36,73.03 94.78,73.01 IC7.3 | 83.39,82.89 v83.39,83.16 | v8.31,77.44 8.22,78.08 IC1.29 | v18.47,26.66 24.33,20.79 24.49,20.79 CF1.21
  Route2 0.178: v88.38,81.86 87.69,81.86 86.4,83.16 v83.39,83.16
  Bottom 0.178: v65.44,70.17 66.28,71.01 v66.28,82.6 | v92.83,73.79 92.8,74.32 92.8,77.65 88.58,81.86 v88.38,81.86 | v7.42,81.37 7.42,81.08 7.36,81.03 7.37,79.83 7.37,78.38 v8.31,77.44 8.29,77.1 8.29,36.83 v18.47,26.66
EMA0  (via drill 0.38)
  Top 0.178: v72.2,72.11 72.54,72.45 80,72.45 IC6.3
  Bottom 0.178: v72.2,72.11 72.2,72.02 72.31,71.86 72.17,53.03 72.17,53.01 72.17,52.97 71.17,51.97 70.14,51.97 70.14,24.28 70.85,23.57 SBC.35
EMA1  (via drill 0.38)
  Top 0.178: v75.23,55.12 74.7,54.58 v70.59,54.58 | v77.86,74.02 IC6.2
  Bottom 0.178: v77.86,74.02 77.33,73.48 77.33,57.21 v75.23,55.12 | v70.59,54.58 69.79,53.78 69.79,17.02 70.85,15.95 SBC.41
EMA2  (via drill 0.38)
  Top 0.178: v79.43,74.66 79.65,74.66 80,75.01 IC6.1
  Bottom 0.178: v79.43,74.66 77.71,72.95 77.71,55.19 74.49,51.97 72.32,51.97 72.32,42.25 71.42,41.36 SBC.21
FLASH_L
  Top 0.178: IC6.14 86.17,73.06 85.9,73.33 79.85,73.33 79.81,73.29 70.05,73.29 69.86,73.3 69.82,73.36 69.69,73.36 39.19,73.36 38.86,73.69 28.71,73.69 28.47,73.7 25.39,76.76 23.99,76.76 18.89,71.65 6.81,71.65 6.81,78.05 IC1.26
FLASH_RDY  (via drill 0.38)
  Top 0.178: v13.28,95.5 10.73,95.5 10.73,97.26 IC1.15 | v24.26,76.11 27.03,73.37 27.18,73.37 27.19,73.36 38.36,73.36 38.58,73.14 39.27,72.45 70.89,72.45 71.88,71.46 79.24,71.46 79.85,72.07 82.89,72.07 84.15,70.82 90.02,70.82 91.5,69.33 93.9,69.33 IC7.6
  Bottom 0.178: v13.28,95.5 24.26,84.53 v24.26,76.11
FPGA_DONE_H  (via drill 0.38)
  Top 0.178: v116.69,58.86 114.53,58.86 112.69,57.03 IC12.72 | v98.53,73.36 97.86,74.03 95.69,74.03 IC7.2
  Route2 0.178: v116.69,58.86 116.69,62.19 105.53,73.36 v98.53,73.36
FPGA_INIT_L/RTC_CLK  (via drill 0.38)
  Top 0.178: IC12.68 110.48,55.12 111.32,55.12 113.18,56.98 113.64,56.98 J3.1 | v119.28,20.56 121.91,20.56 122.29,20.18 IC16.7 | v92.86,71.86 95.36,71.86 95.53,71.69 IC7.4 | v93.86,65.19 94.53,65.19 94.53,63.36 R3.2
  Route2 0.178: v92.86,71.86 94.36,71.86 95.19,72.69 101.69,72.69 113.03,61.36 113.53,61.36 114.03,60.86 114.03,58.36 115.03,57.36 J3.1 | v93.86,65.19 93.19,65.19 92.19,66.19 v91.69,66.19
  Bottom 0.178: v119.28,20.56 116.42,23.42 116.42,56.95 J3.1 | v91.69,66.19 91.03,66.86 91.03,69.03 92.03,70.03 92.03,71.19 92.69,71.86 v92.86,71.86
FPGA_L  (via drill 0.38)
  Top 0.178: v118.4,38.54 118.02,38.16 111.58,38.16 109.11,35.69 105.33,35.69 105.33,36.91 IC12.31 | v91.77,68.68 91.05,67.96 88.15,67.96 IC6.10
  Route2 0.178: v113.14,60.72 101.6,72.26 95.35,72.26 v91.77,68.68
  Bottom 0.178: v118.4,38.54 117.68,39.27 117.68,44.3 117.72,44.34 117.72,44.91 117.68,44.95 117.68,52.22 117.79,52.34 117.79,56.64 115.58,58.85 113.14,58.85 v113.14,60.72
FPGA_PROGRAM_L  (via drill 0.38)
  Top 0.178: v103.85,53.4 105.3,53.4 107.35,55.46 108.92,55.46 IC12.69 | v101.26,53.06 101.26,56.87 101.41,56.87 101.79,57.25 101.79,58.09 IC12.85 101.9,59.65 101.9,59.99 102.74,60.83 103.09,60.83 103.09,61.79 102.67,62.2 102.13,62.2 102.1,62.17 100.65,62.17 100.19,62.62 R2.2
  Bottom 0.178: v103.85,53.4 102.82,53.4 102.48,53.06 v101.26,53.06
FPGA_WR_L/RTC_IO  (via drill 0.38)
  Top 0.178: v105.18,39.04 104.91,39.04 104.91,38.47 IC12.30 | R7.2 112.57,36.53 v113.14,36.53 113.49,36.37 113.64,36.37 v114.44,35.57 | v117.72,21.21 122.59,21.21 123.58,20.22 IC16.6
  Route2 0.178: v105.18,39.04 105.45,39.04 107.96,36.53 v113.14,36.53
  Bottom 0.178: v117.72,21.21 114.44,24.49 v114.44,35.57
G0  (via drill 0.38)
  Top 0.178: v104.46,45.52 102.25,45.52 100.38,47.38 93.22,47.38 92.11,48.49 89.26,48.49 IC12.126 | v112.19,40.3 112.31,40.18 117.34,40.18 118.25,39.27 127.13,39.27 127.28,39.42 129.45,39.42 v131.39,41.36 | v138.71,62.24 140.31,63.84 RN2.2
  Route2 0.178: v104.46,45.52 105.37,45.52 110.59,40.3 v112.19,40.3
  Bottom 0.178: v131.39,41.36 138.71,48.68 v138.71,62.24
GND  (via drill 0.38)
